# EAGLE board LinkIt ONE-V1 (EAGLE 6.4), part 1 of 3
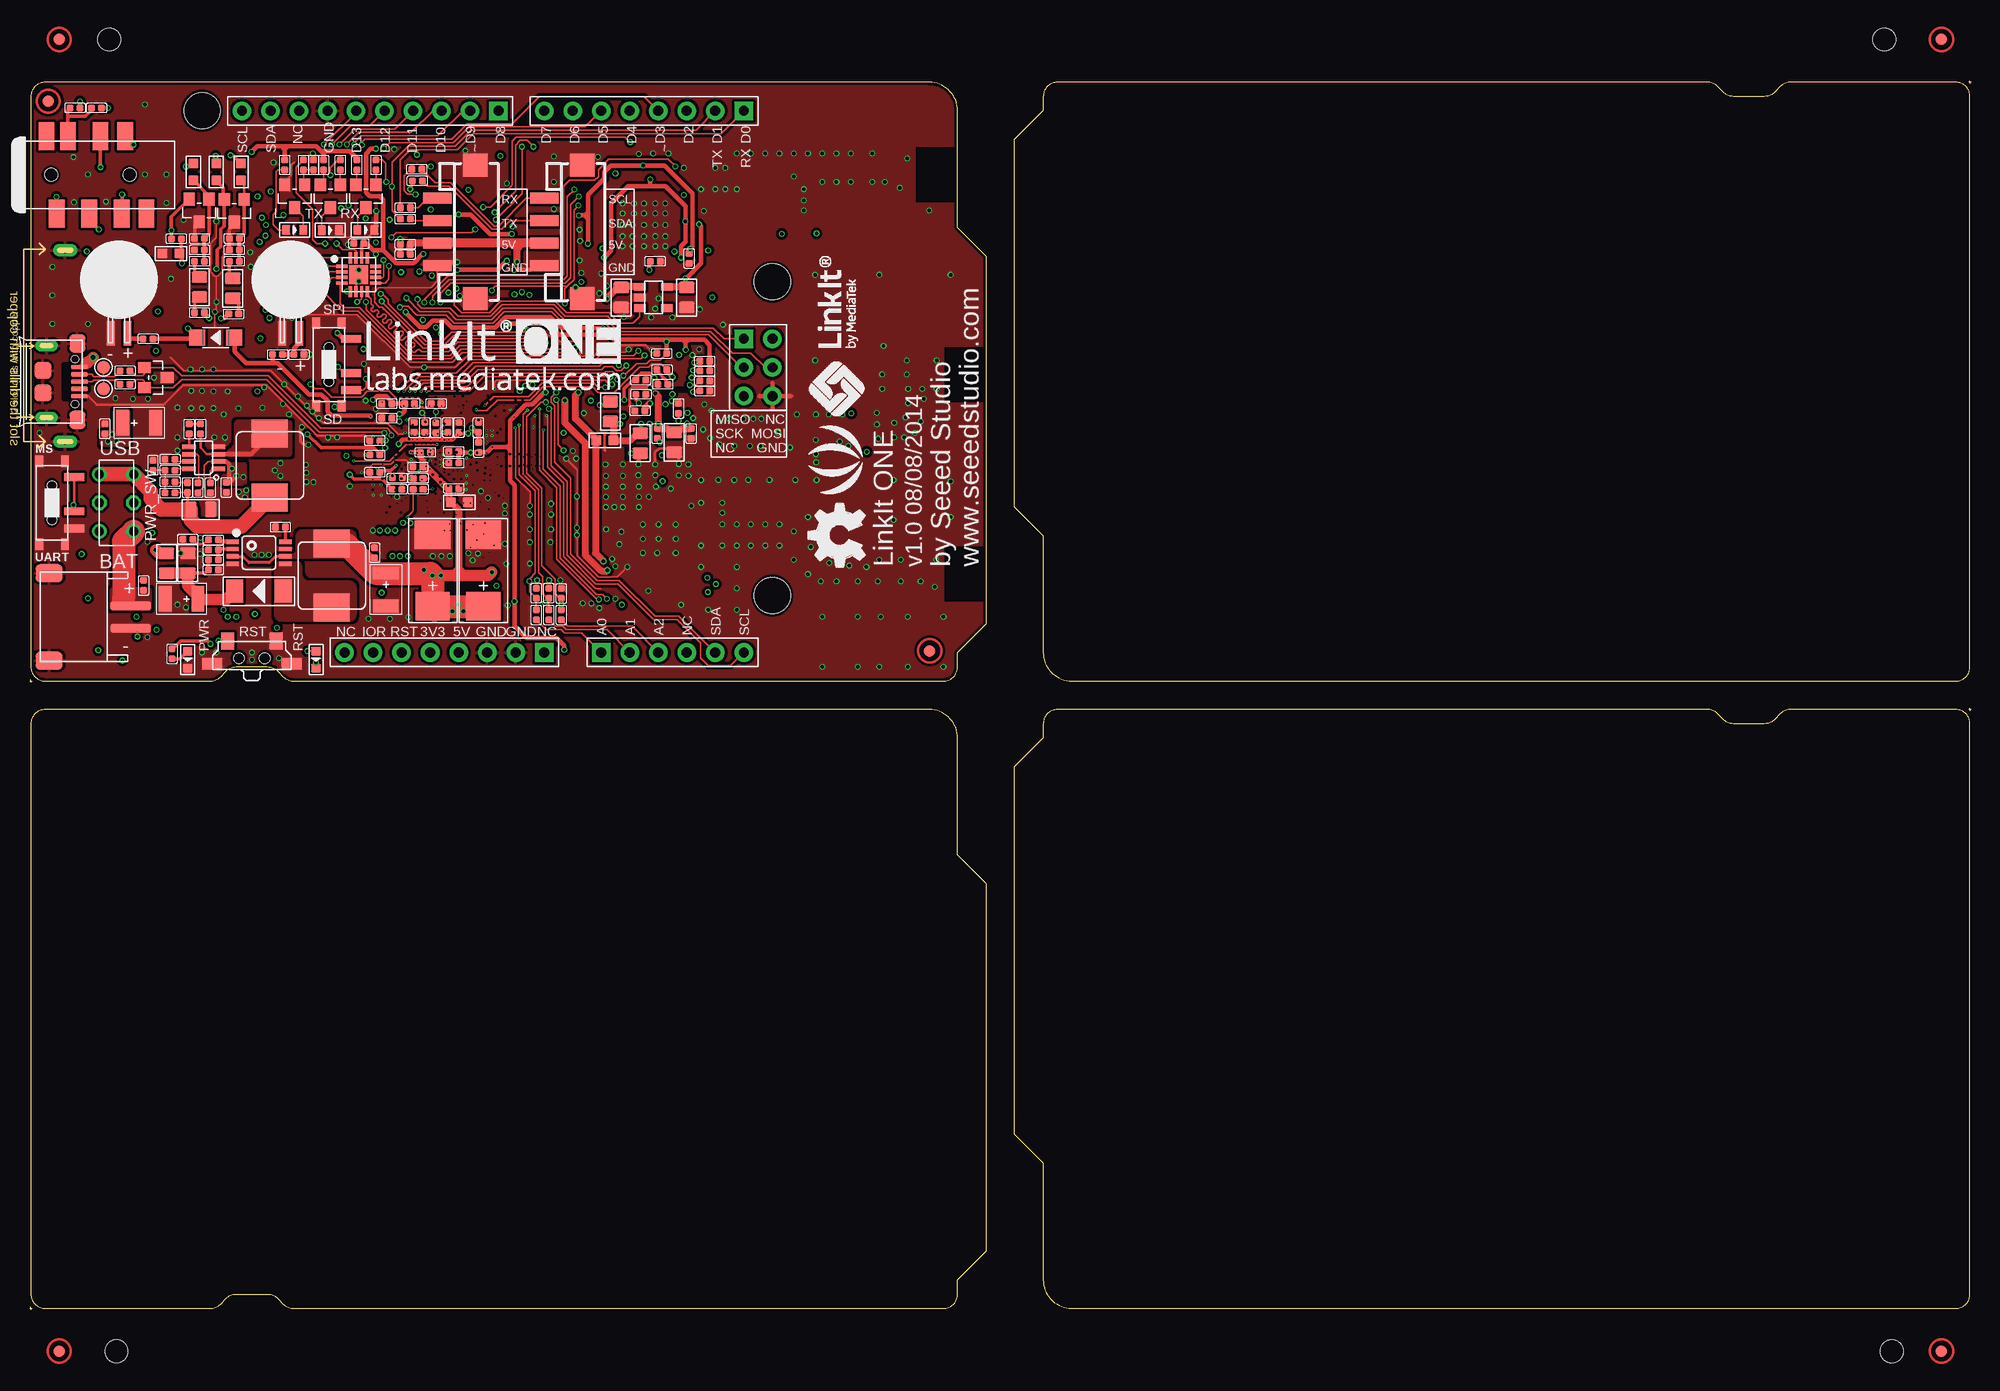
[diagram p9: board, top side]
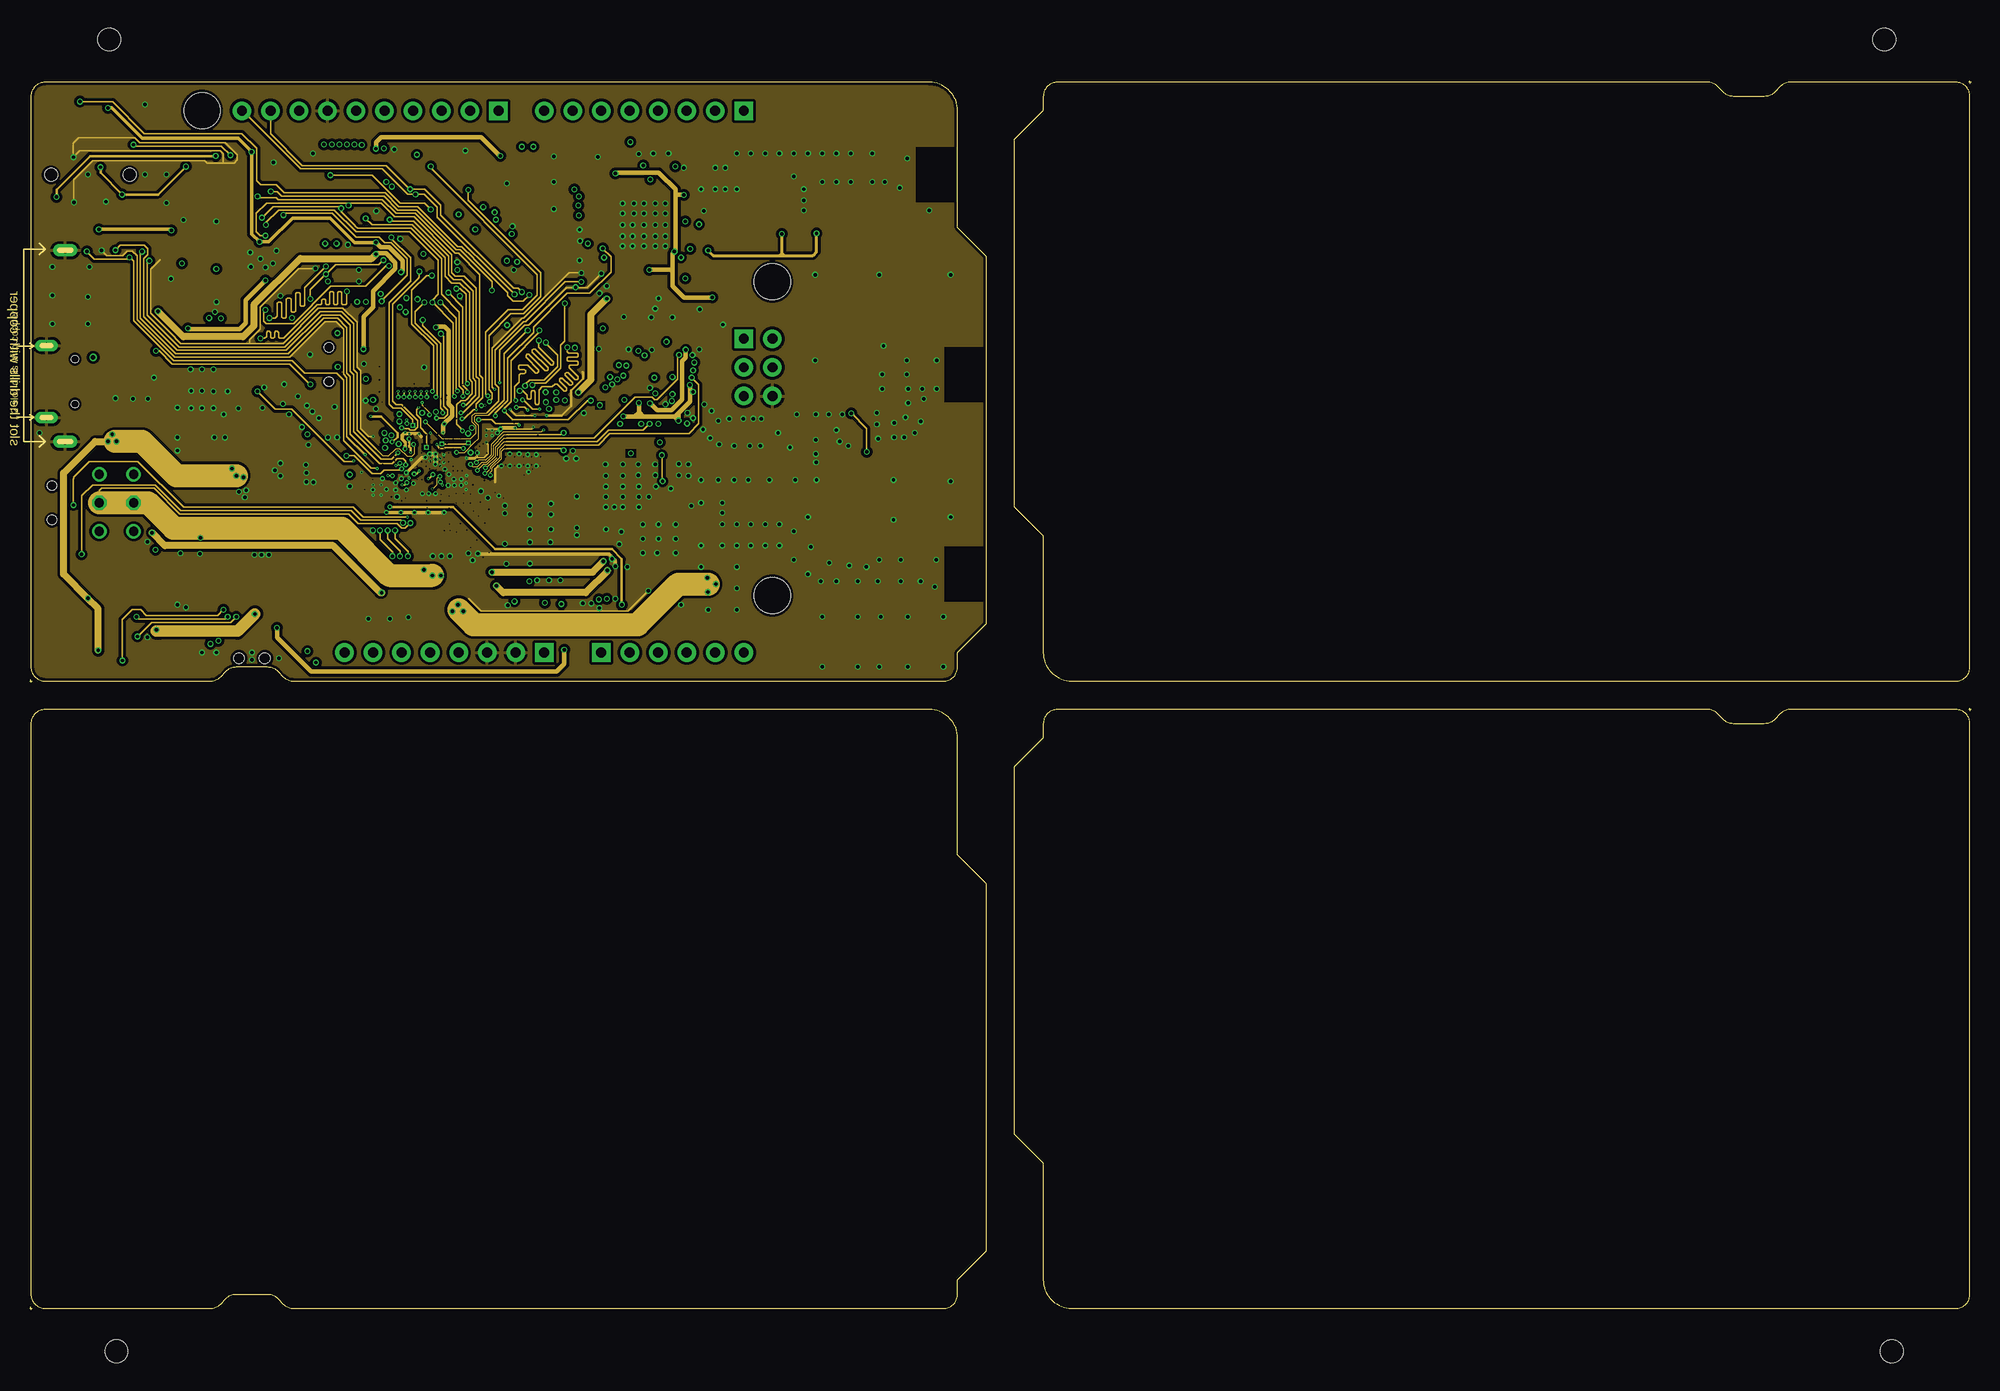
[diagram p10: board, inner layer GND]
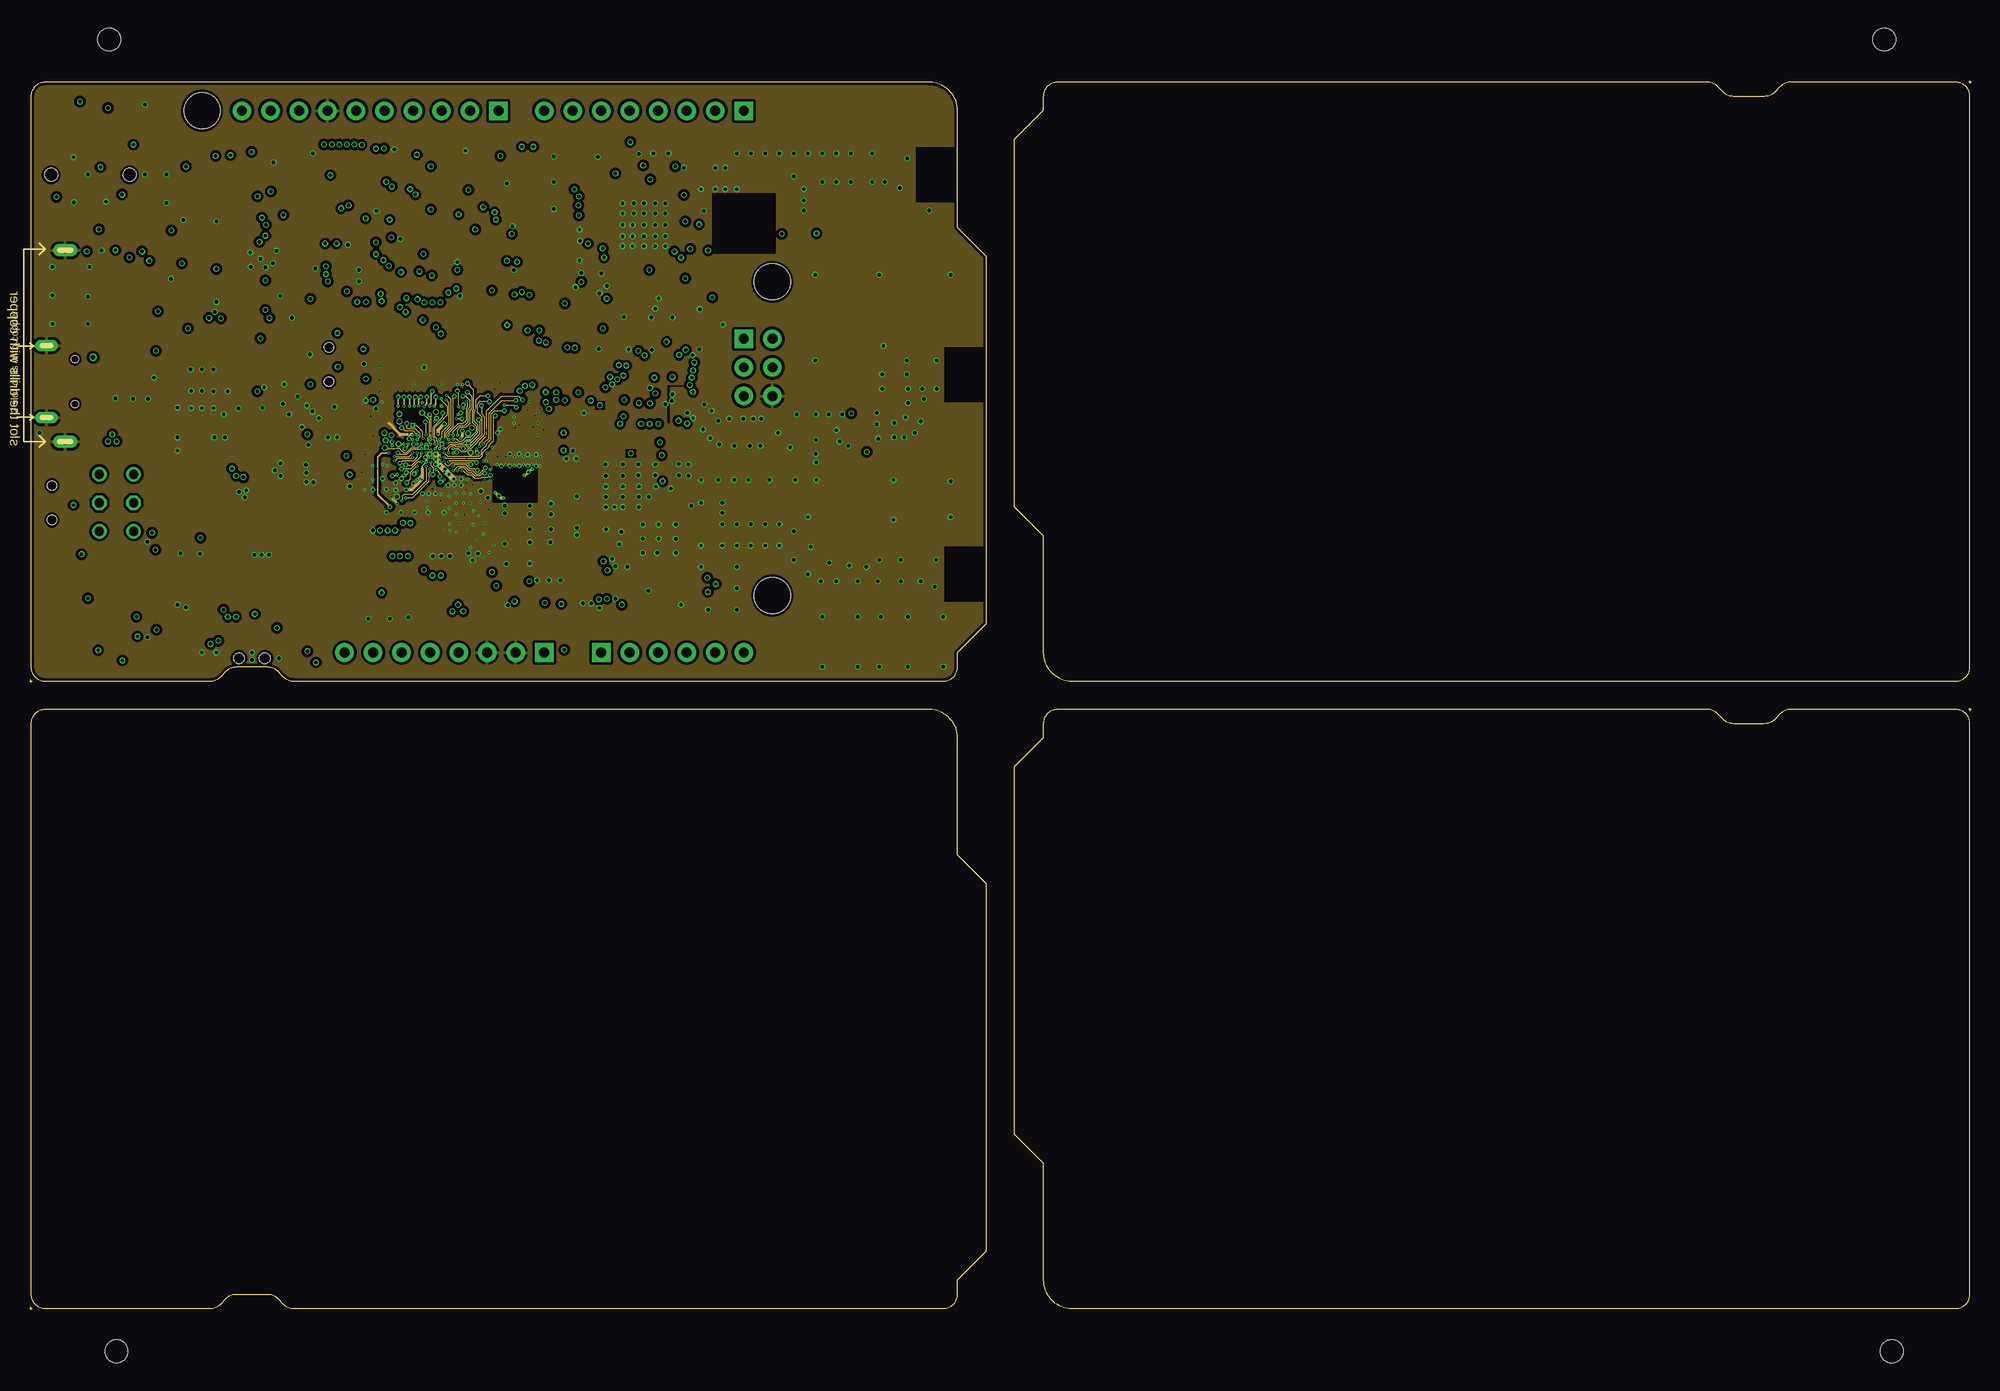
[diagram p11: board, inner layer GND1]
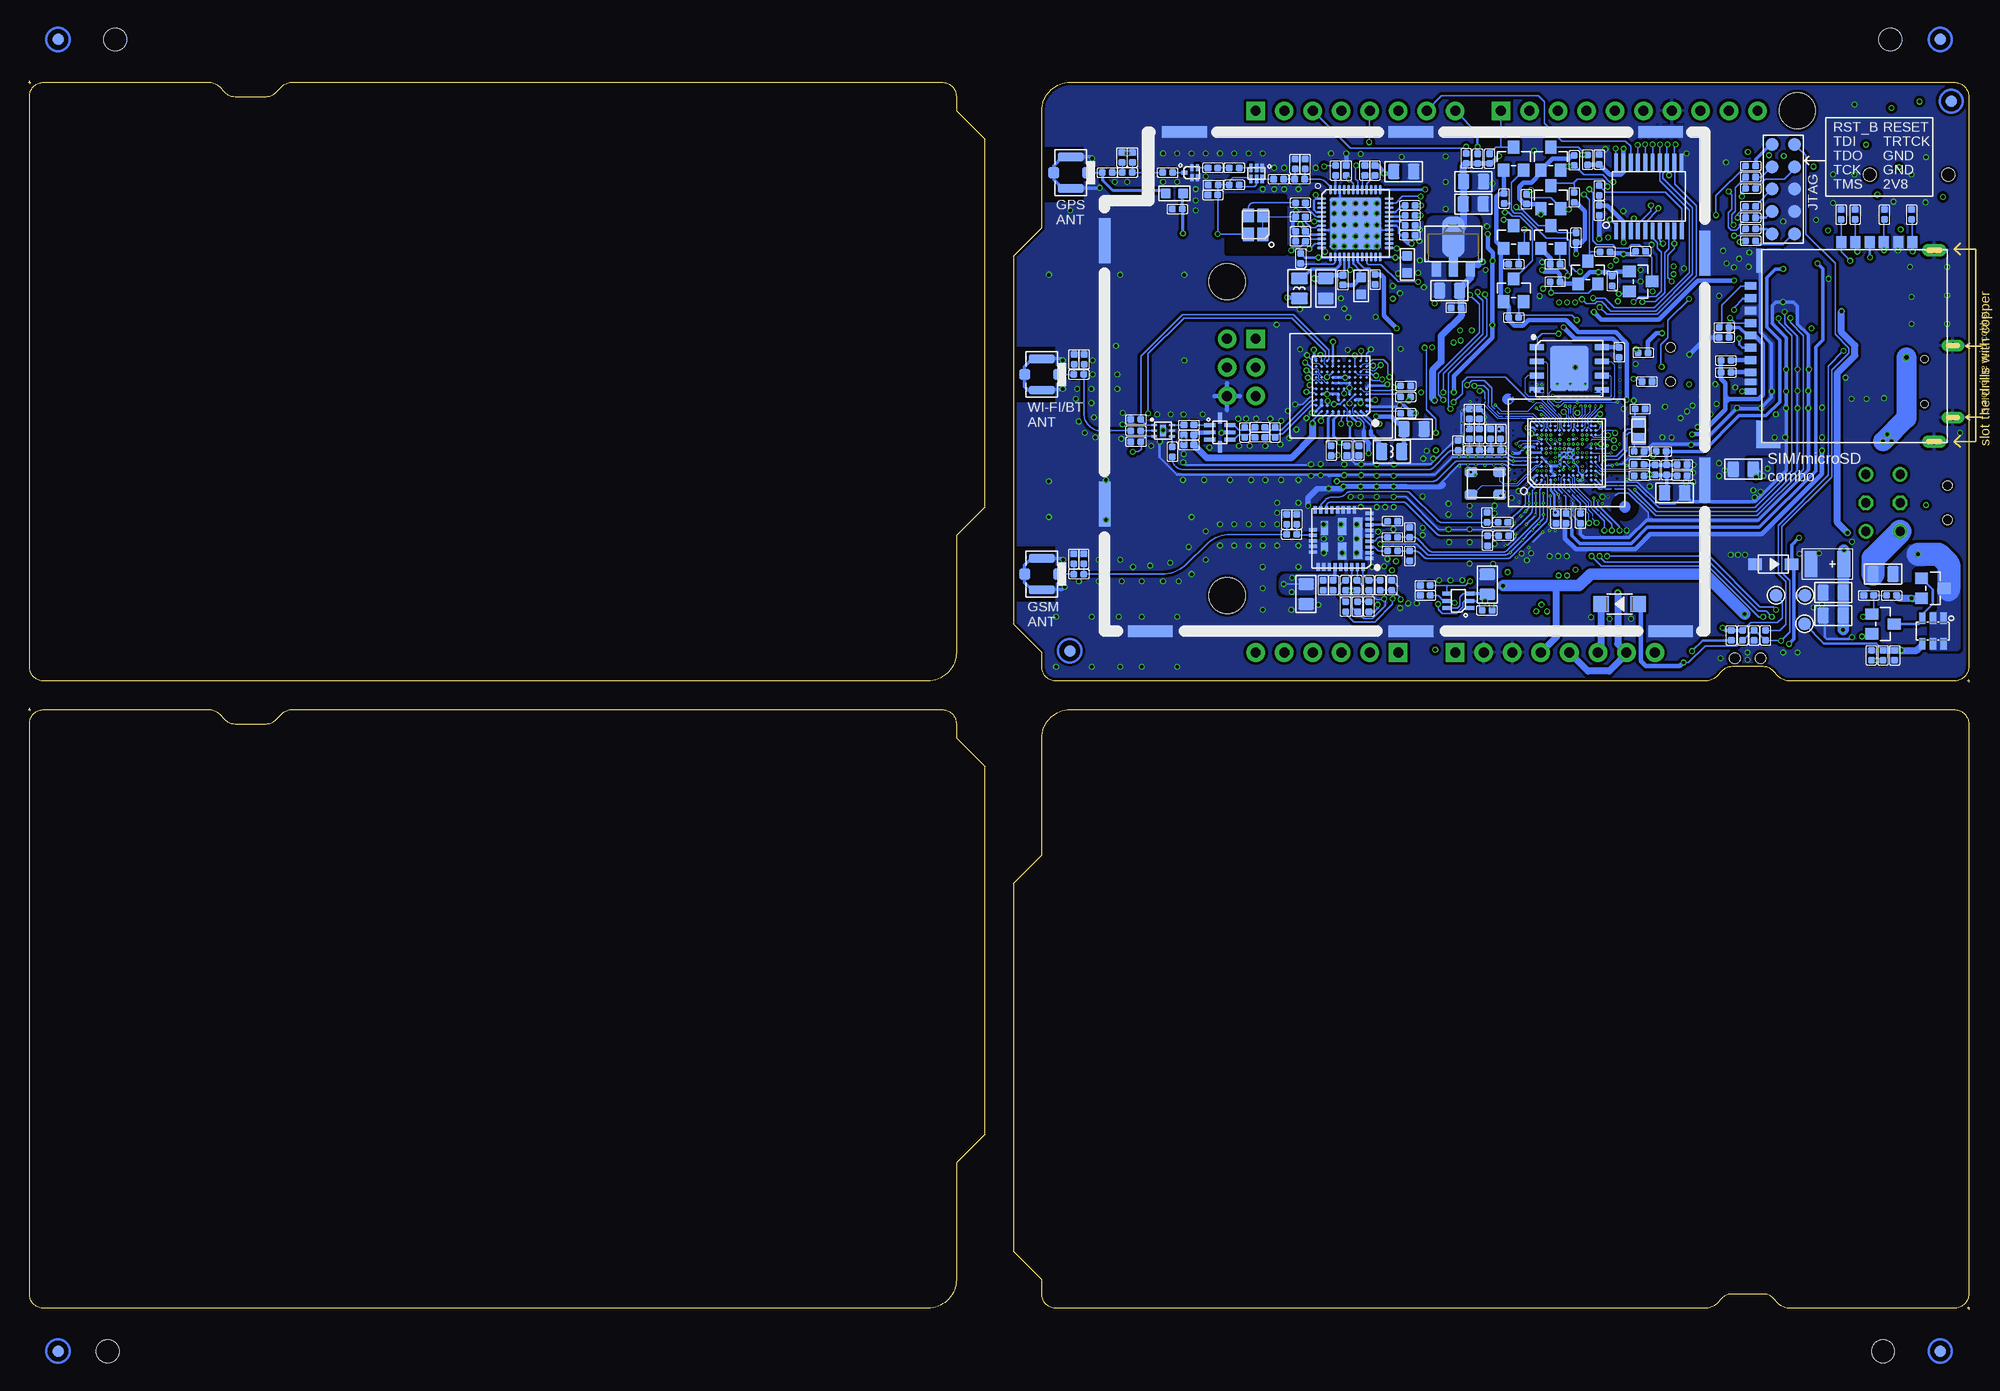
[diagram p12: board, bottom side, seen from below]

Size 172.97 x 109.47 mm. Coordinates in mm from the lower left corner, seen from the top.
Outline: 96 segments
Copper layers [2:(1+(2*15)+16):15]: Top 0.035mm / dielectric 0.2mm / GND 0.0175mm / dielectric 0.7mm / GND1 0.0175mm / dielectric 0.2mm / Bottom 0.035mm
Design rules "default *": minimum track width 3mil, minimum drill 4mil, track to track 3mil, track to pad 3mil, pad to pad 3mil, via to via 3mil, smd to smd 0mil, copper to edge 10mil, drill to drill 8mil, minimum pad ring 2mil, minimum via ring 2mil, stop-mask expansion 2mil, vias tented up to drill 25mil, thermal gap 10mil
Net classes: 0 default: width 0.076 mm, drill 0.102 mm, clearance 0.076 mm
Holes 2.03 mm at 7.11,113.16 165.23,113.16 165.86,-3.68 7.75,-3.68
tRestrict: area 53.2,75.8 to 55.1,76.8; area 56.4,80.4 to 56.9,80.9; area 57,81.3 to 57.5,81.8; area 58.4,79.6 to 58.9,80.1; area 50.5,80.4 to 52.5,81.4; area 65.4,80.6 to 67,82.2; 4 lines
bRestrict: area 61.1,94.1 to 66.2,99.2; area 41.4,72.1 to 45,75.1; area 53,75.8 to 54,76.8; area 57,81.3 to 57.5,81.8; area 55.8,80.3 to 58,81.8; area 65.4,80.6 to 67,82.2; 4 lines

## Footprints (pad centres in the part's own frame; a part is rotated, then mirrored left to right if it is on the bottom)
C0805 = smd 1.016 x 1.397: 1 -0.889,0; 2 0.889,0
C0402 = smd 0.635 x 0.635: 1 -0.445,0; 2 0.445,0
AVX-D = smd 2.54 x 3.048: + -3.175,0 | smd 2.54 x 3.175: - 3.175,0
C0603 = smd 0.889 x 0.889: 1 -0.762,0; 2 0.762,0
AVX-B = smd 1.143 x 2.286: + -1.46,0; - 1.46,0
2P-D6.8MMX1.8MMH = smd 2.2 x 0.7: + 4.8,0.75; - 4.8,-0.75
SOD123 = smd 1.397 x 1.397: + -1.651,0; - 1.651,0
SOD123-2.7X1.6 = smd 1.2 x 1.02: 1 -1.635,0; 2 1.635,0
SOT23 = smd 1.016 x 1.143: 1 -0.889,-1.016; 2 0.889,-1.016; 3 0,1.016
D2010 = smd 1.524 x 2.032: + -2.159,0; - 2.159,0
TP_4545 = smd 1.143 x 1.143: T 0,0
4P-U-FL = smd 1.016 x 1.016: D -1.524,0; GND3 1.524,0 | smd 2.286 x 0.762: GND1 0,1.397; GND2 0,-1.397
4P-SMD-2.0 = smd 0.965 x 2.54: 1 -3,0; 2 -1,0; 3 1,0; 4 3,0 | smd 2.032 x 2.184: SS1 -5.946,3.4; SS2 5.946,3.4
JST-SMD-2.0-90D = smd 1.6 x 2.4: 3 3.9,-2.181; 4 -3.9,-2.181 | smd 0.8 x 3.6: + -1,5.08; - 1,5.08
16P-L17.4MM*W16.5MM*H2.7MM = smd 0.7 x 1: 1 -2.35,9.25; 2 -1.25,9.25; 3 -0.15,9.25; 4 0.95,9.25; 5 2.05,9.25; 6 3.15,9.25; 7 4.25,9.25; 8 5.35,9.25 | smd 1.1 x 0.9: C1 9.25,-5.16; C2 9.25,-2.62; C3 9.25,-0.08; C5 9.25,-3.89; C6 9.25,-1.35; C7 9.25,1.19 | drill 0.5 pad 1.1 long: P1 -8.525,-7.1; P2 8.525,-7.1 | smd 0.5 x 1.65: P3 -8.85,7.425 | smd 2.45 x 0.5: P4 -7.875,8.5 | smd 2.13 x 0.5: P5 7.585,8.5 | smd 0.6 x 1: SA -4.05,9.25; SB -3.2,9.25
MICRO-USB = smd 0.381 x 1.524: 1 -1.3,-0.25; 2 -0.65,-0.25; 3 0,-0.25; 4 0.65,-0.25; 5 1.3,-0.25 | smd 1.6 x 1.397: S1 -3.4,-0.427; S6 3.4,-0.427 | drill 0.508 pad 1.016 long: S2 -3.226,-3.175; S5 3.226,-3.175 | smd 1.5 x 1.5: S3 -1,-3.5; S4 1,-3.5 | hole 0.635: -2,-0.65; 2,-0.65
8P-3.5-SMD = smd 1.4 x 2.5: 1 2.8,-3.45; 2 5.7,-3.45; 3 8.6,-3.45; 4 8.9,3.45; 5 1.9,3.45; 6 3.8,3.45; 7 6.7,3.45; 8 10.8,-3.45 | hole 1.149: 2.3,0; 9.3,0
2*5P-2.0-TESTPOINT = smd 1.143 x 1.143: 1 -1,4; 2 -1,2; 3 -1,0; 4 -1,-2; 5 -1,-4; 6 1,-4; 7 1,-2; 8 1,0; 9 1,2; 10 1,4
LED-0603 = smd 0.762 x 0.889: + -0.762,0; - 0.762,0
L0402 = smd 0.635 x 0.635: 1 -0.445,0; 2 0.445,0
L0603 = smd 0.889 x 0.889: 1 -0.762,0; 2 0.762,0
0806 = smd 1.016 x 1.524: 1 -0.889,0; 2 0.889,0
L0630 = smd 2.5 x 3.2: 1 -2.85,0; 2 2.85,0
L0805 = smd 1.016 x 1.397: 1 -0.889,0; 2 0.889,0
ROUND-MARK-1.0 = smd 1.016 x 1.016: P$1 0,0
R0402 = smd 0.635 x 0.635: 1 -0.445,0; 2 0.445,0
R0805 = smd 1.016 x 1.397: 1 -0.889,0; 2 0.889,0
4P-SMD-7X3.5X3.5H = smd 1.143 x 1.524: 1 -2.159,1.524; 2 2.159,1.524 | smd 1.778 x 1.016: S1 -3.556,-0.508; S2 3.556,-0.508 | hole 0.95: -1.15,0; 1.15,0
3P-SMD-2CH-6.6X2.8-REINFORCE = smd 1.8 x 0.7: A 1.978,2.286; B 1.978,-2.286; COM 1.978,-0.762 | smd 0.7 x 1.016: SS1 -1.15,-3.683; SS2 1.15,-3.683; SS3 1.15,3.683; SS4 -1.15,3.683 | hole 0.813: 0,-1.524; 0,1.524
6P-2CH-2.54-7.6X3.0 = drill 0.813 pad 1.27: CH1A -1.524,2.54; CH1B -1.524,-2.54; CH2A 1.524,2.54; CH2B 1.524,-2.54 | drill 0.813 pad 1.27 octagon: COM1 -1.524,0; COM2 1.524,0
TFBGA84 = smd 0.25 x 0.25: A1 -2.25,2.25; A2 -1.75,2.25; A3 -1.25,2.25; A4 -0.75,2.25; A5 -0.25,2.25; A6 0.25,2.25; A7 0.75,2.25; A8 1.25,2.25; A9 1.75,2.25; A10 2.25,2.25; B1 -2.25,1.75; B3 -1.25,1.75; B5 -0.25,1.75; B8 1.25,1.75; B9 1.75,1.75; B10 2.25,1.75; C1 -2.25,1.25; C2 -1.75,1.25; C3 -1.25,1.25; C5 -0.25,1.25; C6 0.25,1.25; C9 1.75,1.25; C10 2.25,1.25; D1 -2.25,0.75; D2 -1.75,0.75; D3 -1.25,0.75; D4 -0.75,0.75; D6 0.25,0.75; D7 0.75,0.75; D9 1.75,0.75; D10 2.25,0.75; E1 -2.25,0.25; E2 -1.75,0.25; E3 -1.25,0.25; E5 -0.25,0.25; E6 0.25,0.25; E7 0.75,0.25; E8 1.25,0.25; E9 1.75,0.25; E10 2.25,0.25; F2 -1.75,-0.25; F3 -1.25,-0.25; F4 -0.75,-0.25; F6 0.25,-0.25; F7 0.75,-0.25; F8 1.25,-0.25; F9 1.75,-0.25; F10 2.25,-0.25; G1 -2.25,-0.75; G2 -1.75,-0.75; G3 -1.25,-0.75; G4 -0.75,-0.75; G6 0.25,-0.75; G7 0.75,-0.75; G9 1.75,-0.75; G10 2.25,-0.75; H1 -2.25,-1.25; H2 -1.75,-1.25; H3 -1.25,-1.25; H4 -0.75,-1.25; H5 -0.25,-1.25; H6 0.25,-1.25; H7 0.75,-1.25; H8 1.25,-1.25; H9 1.75,-1.25; H10 2.25,-1.25; J1 -2.25,-1.75; J2 -1.75,-1.75; J3 -1.25,-1.75; J4 -0.75,-1.75; J5 -0.25,-1.75; J6 0.25,-1.75; J7 0.75,-1.75; J8 1.25,-1.75; J9 1.75,-1.75; J10 2.25,-1.75; K1 -2.25,-2.25; K2 -1.75,-2.25; K4 -0.75,-2.25; K6 0.25,-2.25; K7 0.75,-2.25; K8 1.25,-2.25; K9 1.75,-2.25; K10 2.25,-2.25
QFN48-6X6MM = smd 0.25 x 0.8: 1 -2.2,-3; 2 -1.8,-3; 3 -1.4,-3; 4 -1,-3; 5 -0.6,-3; 6 -0.2,-3; 7 0.2,-3; 8 0.6,-3; 9 1,-3; 10 1.4,-3; 11 1.8,-3; 12 2.2,-3; 25 2.2,3; 26 1.8,3; 27 1.4,3; 28 1,3; 29 0.6,3; 30 0.2,3; 31 -0.2,3; 32 -0.6,3; 33 -1,3; 34 -1.4,3; 35 -1.8,3; 36 -2.2,3 | smd 0.8 x 0.25: 13 3,-2.2; 14 3,-1.8; 15 3,-1.4; 16 3,-1; 17 3,-0.6; 18 3,-0.2; 19 3,0.2; 20 3,0.6; 21 3,1; 22 3,1.4; 23 3,1.8; 24 3,2.2; 37 -3,2.2; 38 -3,1.8; 39 -3,1.4; 40 -3,1; 41 -3,0.6; 42 -3,0.2; 43 -3,-0.2; 44 -3,-0.6; 45 -3,-1; 46 -3,-1.4; 47 -3,-1.8; 48 -3,-2.2 | smd 4.6 x 4.6: PAD 0,0
WSON8-6X5X0.8H-W/HEAT = smd 0.5 x 1.25: 1 -1.905,-2.875; 2 -0.635,-2.875; 3 0.635,-2.875; 4 1.905,-2.875; 5 1.905,2.875; 6 0.635,2.875; 7 -0.635,2.875; 8 -1.905,2.875 | smd 4 x 3.4: PAD 0,0
SOT-25J = smd 0.7 x 1: 1 -0.95,-1.2; 2 0,-1.2; 3 0.95,-1.2; 4 0.95,1.2; 5 -0.95,1.2
TQFN16 = smd 1 x 0.3: 1 -1.5,0.75; 2 -1.5,0.25; 3 -1.5,-0.25; 4 -1.5,-0.75; 9 1.5,-0.75; 10 1.5,-0.25; 11 1.5,0.25; 12 1.5,0.75 | smd 0.3 x 1: 5 -0.75,-1.5; 6 -0.25,-1.5; 7 0.25,-1.5; 8 0.75,-1.5; 13 0.75,1.5; 14 0.25,1.5; 15 -0.25,1.5; 16 -0.75,1.5 | smd 1.7 x 1.7: PAD 0,0
VFBGA143 = smd 0.25 x 0.25: A1 -2.4,2.6; A2 -2,2.6; A3 -1.6,2.6; A5 -0.8,2.6; A6 -0.4,2.6; A8 0.4,2.6; A9 0.8,2.6; A11 1.6,2.6; A12 2,2.6; A13 2.4,2.6; B1 -2.4,2.2; B2 -2,2.2; B3 -1.6,2.2; B4 -1.2,2.2; B5 -0.8,2.2; B6 -0.4,2.2; B7 0,2.2; B8 0.4,2.2; B9 0.8,2.2; B10 1.2,2.2; B11 1.6,2.2; B12 2,2.2; B13 2.4,2.2; C2 -2,1.8; C3 -1.6,1.8; C4 -1.2,1.8; C5 -0.8,1.8; C7 0,1.8; C8 0.4,1.8; C11 1.6,1.8; C12 2,1.8; D1 -2.4,1.4; D2 -2,1.4; D3 -1.6,1.4; D4 -1.2,1.4; D5 -0.8,1.4; D7 0,1.4; D8 0.4,1.4; D10 1.2,1.4; D11 1.6,1.4; D12 2,1.4; D13 2.4,1.4; E1 -2.4,1; E2 -2,1; E5 -0.8,1; E6 -0.4,1; E7 0,1; E8 0.4,1; E9 0.8,1; E12 2,1; E13 2.4,1; F2 -2,0.6; F3 -1.6,0.6; F4 -1.2,0.6; F5 -0.8,0.6; F6 -0.4,0.6; F7 0,0.6; F8 0.4,0.6; F9 0.8,0.6; F10 1.2,0.6; F11 1.6,0.6; F12 2,0.6; G1 -2.4,0.2; G2 -2,0.2; G4 -1.2,0.2; G5 -0.8,0.2; G6 -0.4,0.2; G7 0,0.2; G8 0.4,0.2; G9 0.8,0.2; G12 2,0.2; G13 2.4,0.2; H1 -2.4,-0.2; H2 -2,-0.2; H5 -0.8,-0.2; H6 -0.4,-0.2; H7 0,-0.2; H8 0.4,-0.2; H9 0.8,-0.2; H10 1.2,-0.2; H12 2,-0.2; H13 2.4,-0.2; J2 -2,-0.6; J3 -1.6,-0.6; J4 -1.2,-0.6; J5 -0.8,-0.6; J6 -0.4,-0.6; J7 0,-0.6; J8 0.4,-0.6; J9 0.8,-0.6; J10 1.2,-0.6; J11 1.6,-0.6; J12 2,-0.6; K1 -2.4,-1; K2 -2,-1; K5 -0.8,-1; K6 -0.4,-1; K7 0,-1; K8 0.4,-1; K9 0.8,-1; K12 2,-1; K13 2.4,-1; L1 -2.4,-1.4; L2 -2,-1.4; L3 -1.6,-1.4; L4 -1.2,-1.4; L6 -0.4,-1.4; L7 0,-1.4; L9 0.8,-1.4; L10 1.2,-1.4; L11 1.6,-1.4; L12 2,-1.4; L13 2.4,-1.4; M2 -2,-1.8; M3 -1.6,-1.8; M6 -0.4,-1.8; M7 0,-1.8; M10 1.2,-1.8; M11 1.6,-1.8; M12 2,-1.8; N1 -2.4,-2.2; N2 -2,-2.2; N3 -1.6,-2.2; N4 -1.2,-2.2; N5 -0.8,-2.2; N6 -0.4,-2.2; N7 0,-2.2; N8 0.4,-2.2; N9 0.8,-2.2; N10 1.2,-2.2; N11 1.6,-2.2; N12 2,-2.2; N13 2.4,-2.2; P1 -2.4,-2.6; P2 -2,-2.6; P3 -1.6,-2.6; P5 -0.8,-2.6; P6 -0.4,-2.6; P8 0.4,-2.6; P9 0.8,-2.6; P11 1.6,-2.6; P12 2,-2.6; P13 2.4,-2.6
SOT23-6L = smd 0.55 x 1.016: 1 -0.95,-1.143; 2 0,-1.143; 3 0.95,-1.143; 4 0.95,1.143; 5 0,1.143; 6 -0.95,1.143
5P-SMD-1.4X1.1MM = smd 0.55 x 0.326: 1 -0.65,0 | smd 0.25 x 0.625: 2 0,-0.438; 3 0.5,-0.438; 4 0.5,0.438; 5 0,0.438
SHIELD-SMD-44.5X53.5 = smd 4 x 1.016: 1 3.937,0; 4 49.403,44.45; 5 46.355,0; 6 3.048,44.45; 9 26.162,44.45; 10 26.162,0 | smd 1.016 x 4: 2 0,30.988; 3 53.467,9.652; 7 53.467,33.147; 8 0,10.795
ARDUINO-38P = drill 0.889 pad 1.651 square: 1 63.5,50.8; 9 41.656,50.8; 19 50.8,2.54; 25 45.72,2.54; 38 63.5,30.48 | drill 0.889 pad 1.651: 2 60.96,50.8; 3 58.42,50.8; 4 55.88,50.8; 5 53.34,50.8; 6 50.8,50.8; 7 48.26,50.8; 8 45.72,50.8; 10 39.116,50.8; 11 36.576,50.8; 12 34.036,50.8; 13 31.496,50.8; 14 28.956,50.8; 15 26.416,50.8; 16 23.876,50.8; 17 21.336,50.8; 18 18.796,50.8; 20 53.34,2.54; 21 55.88,2.54; 22 58.42,2.54; 23 60.96,2.54; 24 63.5,2.54; 26 43.18,2.54; 27 40.64,2.54; 28 38.1,2.54; 29 35.56,2.54; 30 33.02,2.54; 31 30.48,2.54; 32 27.94,2.54; 33 66.04,30.48; 34 66.04,27.94; 35 66.04,25.4; 36 63.5,25.4; 37 63.5,27.94 | hole 3.2: 15.24,50.8; 66.04,35.56; 66.04,7.62
TSOT23-8 = smd 0.4 x 1.2: 1 -0.975,-1.3; 2 -0.325,-1.3; 3 0.325,-1.3; 4 0.975,-1.3; 5 0.975,1.3; 6 0.325,1.3; 7 -0.325,1.3; 8 -0.975,1.3
6P-SMD-1.5X1.0X0.72H = smd 0.3 x 0.75: 1 -0.5,-0.5; 2 0,-0.5; 3 0.5,-0.5; 4 0.5,0.5; 5 0,0.5; 6 -0.5,0.5
32P-SMD-RF1798-5.3MMX5.25MMX0.73H = smd 0.7 x 0.3: 1 -2.525,1.77; 2 -2.525,1.27; 3 -2.525,0.77; 4 -2.525,0.27; 5 -2.525,-0.23; 6 -2.525,-0.73; 7 -2.525,-1.23; 8 -2.525,-1.73; 9 -2.525,-2.23; 18 2.525,-0.785; 19 2.525,-0.285; 20 2.525,0.215; 21 2.525,0.715; 22 2.525,1.215 | smd 0.3 x 0.7: 10 -1.175,-2.55; 11 -0.675,-2.55; 12 -0.175,-2.55; 13 0.325,-2.55; 14 0.825,-2.55; 15 1.325,-2.55; 16 1.825,-2.55; 17 2.325,-2.55; 23 2.055,2.55; 24 1.555,2.55; 25 1.055,2.55; 26 0.555,2.55; 27 0.055,2.55; 28 -0.445,2.55; 29 -0.945,2.55; 30 -1.445,2.55; 31 -1.945,2.55 | smd 0.805 x 3.715: 32 -1.473,0 | smd 0.785 x 1.535: 33 -0.083,1.133; 34 -0.083,-1.055 | smd 0.635 x 0.8: 35 1.493,0.765 | smd 0.635 x 1.245: 36 1.493,-0.933
8P-SMD-2X1.25X0.7H = smd 0.35 x 1: 1 0.65,0.9; 2 0,0.9; 3 -0.65,0.9; 5 -0.65,-0.9; 6 0,-0.9; 7 0.65,-0.9 | smd 1 x 0.35: 4 -1.281,0; 8 1.281,0
TSON6 = smd 0.5 x 0.2: 1 -0.8,0.5; 2 -0.8,0; 3 -0.8,-0.5; 4 0.8,-0.5; 5 0.8,0; 6 0.8,0.5 | smd 0.5 x 1: PAD 0,0
SOT363 = smd 0.35 x 0.8: 1 -0.65,-1.025; 2 0,-1.025; 3 0.65,-1.025; 4 0.65,1.025; 5 0,1.025; 6 -0.65,1.025
TSSOP20 = smd 0.35 x 1.5: 1 -2.925,-3.065; 2 -2.275,-3.065; 3 -1.625,-3.065; 4 -0.975,-3.065; 5 -0.325,-3.065; 6 0.325,-3.065; 7 0.975,-3.065; 8 1.625,-3.065; 9 2.275,-3.065; 10 2.925,-3.065; 11 2.91,3.065; 12 2.26,3.065; 13 1.61,3.065; 14 0.96,3.065; 15 0.325,3.065; 16 -0.325,3.065; 17 -0.975,3.065; 18 -1.625,3.065; 19 -2.275,3.065; 20 -2.925,3.065
SOT89 = smd 0.8 x 1.4: 1 -1.524,-1.905; 3 1.524,-1.905 | smd 0.8 x 1.9: 2 0,-1.651 | smd 2.032 x 3.65: 4 0,0.94
MSOP8 = smd 0.4 x 1.1: 1 -0.975,-2.35; 2 -0.325,-2.35; 3 0.325,-2.35; 4 0.975,-2.35; 5 0.975,2.35; 6 0.325,2.35; 7 -0.325,2.35; 8 -0.975,2.35
2P-SMD-2.05X1.2 = smd 1 x 1.25: 1 -0.75,0; 2 0.75,0
2520 = smd 1.2 x 1: 1 -0.85,-0.65; 2 0.85,-0.65; 3 0.85,0.65; 4 -0.85,0.65
4P-SMD-3.2X2.5 = smd 1.143 x 0.889: 1 -1.27,-1.016; 2 1.27,-1.016; 3 1.27,1.016; 4 -1.27,1.016

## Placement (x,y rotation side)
C1  4.7uF  [C0805]  46.36,90.78 180 bottom
C2  4.7uF  [C0805]  44.22,100.51 0 bottom
C3  100nF  [C0402]  30.73,67.44 90 top
C4  100nF  [C0402]  16.38,65.91 0 top
C5  100nF  [C0402]  33.02,97.92 270 bottom
C6  1uF  [C0402]  50.27,79.86 0 bottom
C7  100nF  [C0402]  33.02,102.46 90 bottom
C8  1uF  [C0402]  37.8,73.15 0 top
C9  1uF  [C0402]  36.2,78.56 270 top
C10  1uF  [C0402]  31.83,79.43 180 top
C11  4.7uF  [C0805]  49.53,78.46 0 bottom
C12  4.7uF  [C0805]  54.41,77.19 270 top
C13  1uF  [C0402]  54.47,81.55 180 top
C14  100nF  [C0402]  54.38,80.09 0 top
C15  1uF  [C0402]  55.5,76.53 270 bottom
C16  1uF  [C0402]  60.15,82.73 180 top
C17  18pF  [C0402]  60.15,81.84 180 top
C18  100nF  [C0402]  58.93,78.05 90 top
C19  100nF  [C0402]  57.81,80.29 270 top
C20  1nF  [C0402]  56.9,76.53 90 bottom
C21  100nF  [C0402]  56.41,82.45 0 top
C22  1uF  [C0402]  54.44,82.83 0 top
C23  1uF  [C0402]  56.31,85.19 180 top
C24  18pF  [C0402]  71.48,101.3 180 bottom
C25  18pF  [C0402]  67.44,101.73 0 bottom
C26  1uF  [C0402]  59.64,95.17 180 bottom
C27  DNP/18pF  [C0402]  75.54,102.64 90 bottom
C28  100nF  [C0402]  33.48,94.92 180 top
C29  1uF  [C0402]  52.98,91.77 270 bottom
C30  SMD CAP Tantalum 470uF-6.3V;D  [AVX-D]  35.92,65.84 90 top
C31  220nF  [C0402]  55.85,91.72 90 bottom
C32  22uF  [C0805]  44.25,98.5 0 bottom
C33  SMD CAP Tantalum 470uF-6.3V;D  [AVX-D]  40.44,65.84 90 top
C34  4.7uF  [C0805]  50.44,101.4 0 bottom
C35  4.7uF  [C0805]  57.38,90.98 270 bottom
C36  1uF  [C0402]  58.75,93.65 270 top
C37  1uF  [C0402]  59.61,93.65 270 bottom
C38  1uF  [C0402]  59.64,97.36 180 bottom
C39  1uF  [C0402]  59.64,96.06 180 bottom
C40  100nF  [C0402]  49.89,95.71 0 bottom
C41  2.2uF  [C0603]  50.11,93.12 270 bottom
C42  DNP/100nF  [C0402]  55.55,101.47 90 bottom
C43  1nF  [C0402]  59.64,98.6 180 bottom
C44  100nF  [C0402]  55.73,93.4 0 top
C45  4.7uF  [C0805]  52.71,90.17 270 top
C46  4.7uF  [C0805]  58.55,90.17 270 top
C47  1uF  [C0402]  37.26,78.59 90 top
C48  1uF  [C0402]  9.02,63.63 180 bottom
C49  SMD CAP Tantalum 47uF-10V;B  [AVX-B]  9.78,78.99 0 top
C50  SMD CAP Tantalum 47uF-10V;B  [AVX-B]  31.75,64.16 270 top
C51  22uF  [C0805]  18.11,90.98 90 top
C52  22uF  [C0805]  15.14,91.11 90 top
C53  390pF  [C0402]  15.14,94.41 180 top
C54  390pF  [C0402]  18.24,94.41 180 top
C55  100nF  [C0402]  29.46,74.3 0 bottom
C56  33pF  [C0402]  25.63,75.29 0 bottom
C57  33pF  [C0402]  25.63,74.3 0 bottom
C58  100nF  [C0402]  29.46,75.31 0 bottom
C59  100pF  [C0402]  28.07,74.8 270 bottom
C60  4.7uF  [C0805]  26.31,72.77 0 bottom
C61  27pF  [C0402]  7.62,97.56 90 bottom
C62  27pF  [C0402]  10.24,97.56 90 bottom
C63  1uF  [C0402]  37.8,76.45 180 top
C64  27pF  [C0402]  11.48,97.56 90 bottom
C65  1uF  [C0402]  5.21,97.56 90 bottom
C66  100nF  [C0402]  21.89,86.61 180 bottom
C67  1.2pF  [C0402]  59.69,100.71 0 bottom
C68  DNP/18pF  [C0402]  60.12,102.06 90 bottom
C69  1uF  [C0402]  38.25,78.59 90 top
C70  1uF  [C0402]  31.83,80.72 180 top
C71  1uF  [C0402]  37.8,75.44 180 top
C72  1uF  [C0402]  35.26,76.38 0 top
C73  2.2uF  [C0603]  38.3,71.93 0 top
C74  22uF  [C0805]  20.19,74.87 180 bottom
C75  22pF  [C0402]  29.39,80.24 0 bottom
C76  22pF  [C0402]  29.46,76.45 0 bottom
C77  100nF  [C0402]  12.52,75.77 180 top
C78  15pF  [C0402]  14.08,73.24 270 top
C79  22uF  [C0805]  15.27,71.3 0 top
C80  18pF  [C0402]  70.61,98.04 180 bottom
C81  330pF  [C0402]  19.23,60.07 270 bottom
C82  DNP/18pF  [C0402]  59.97,70.41 90 bottom
C83  DNP/18pF  [C0402]  60.86,70.41 90 bottom
C84  1.2pF  [C0402]  79.81,84.66 90 bottom
C85  18pF  [C0402]  76.83,101.3 180 bottom
C87  100nF  [C0402]  29.34,94.97 180 top
C88  SMD CAP Tantalum 47uF-10V;B  [AVX-B]  13.54,63.32 180 top
C89  DNP/22pF  [C0402]  47.37,63.8 90 top
C90  100nF  [C0402]  33.48,94.01 180 top
C91  1uF  [C0402]  31.24,85.29 270 bottom
C92  1uF  [C0402]  34.7,70.48 270 bottom
C93  1uF  [C0402]  24,85.09 0 top
C94  1uF  [C0402]  32.77,74.09 0 top
C95  1uF  [C0402]  30.76,76.15 180 top
C96  1uF  [C0402]  30.76,77.42 180 top
C97  100nF  [C0402]  30.76,74.6 180 top
C98  1uF  [C0402]  6.71,78.49 90 top
C99  2.2uF  [C0603]  54.23,91.21 270 bottom
C100  22nF  [C0402]  16.1,73.23 270 top
C101  100nF  [C0402]  34.59,75.08 180 top
C102  DNP/22pF  [C0402]  46.25,63.83 90 top
C103  DNP/22pF  [C0402]  48.51,64.52 180 bottom
C104  1uF  [C0402]  36.88,70.48 270 bottom
C105  100nF  [C0402]  15.24,78.46 90 top
C106  100nF  [C0402]  17.53,73.25 270 top
C107  DNP/EECENOF204Rk  [2P-D6.8MMX1.8MMH]  23.27,91.77 270 top
C108  100nF  [C0402]  45.77,89.26 180 bottom
C109  1uF  [C0402]  10.16,64.52 90 top
C110  1.2pF  [C0402]  45.61,77 90 bottom
C111  1.5pF  [C0402]  44.59,78.02 90 bottom
C112  1.8pF  [C0402]  43.7,79.79 90 bottom
C113  1.5pF  [C0402]  42.68,78.02 90 bottom
C114  0.5pF  [C0402]  41.8,78.02 90 bottom
C115  1.2pF  [C0402]  78.92,84.66 90 bottom
C116  1uF  [C0402]  6.71,58.29 270 bottom
C117  DNP/0.5pF  [C0402]  74.6,102.64 90 bottom
C118  18pF  [C0402]  61.6,100.71 0 bottom
C119  33nF  [C0402]  67.41,100.19 180 bottom
C120  1uF  [C0402]  67.44,99.3 180 bottom
C122  DNP/4.7uF  [C0805]  43,64.62 90 bottom
C124  DNP/18pF  [C0402]  79.83,66.88 90 bottom
C125  DNP/18pF  [C0402]  78.94,66.88 90 bottom
C126  39pF  [C0402]  57.61,64.54 90 bottom
C127  100nF  [C0402]  56.72,64.54 90 bottom
C128  22uF  [C0805]  59.13,63.75 90 bottom
C129  39pF  [C0402]  55.63,64.54 270 bottom
C130  39pF  [C0402]  53.54,64.54 270 bottom
C131  220pF  [C0402]  54.61,64.54 270 bottom
C132  1pF  [C0402]  43.03,70.59 90 bottom
C133  2.7pF  [C0402]  42.98,68.5 270 bottom
C134  2.2pF  [C0402]  49.91,67.14 270 bottom
C135  2.2pF  [C0402]  49.91,69.25 90 bottom
C136  1.5nF  [C0402]  51.44,70.24 0 bottom
C137  18pF  [C0402]  74.3,78.31 0 bottom
C138  18pF  [C0402]  69.57,78.82 0 bottom
C139  1uF  [C0402]  69.57,77.04 180 bottom
C140  10pF  [C0402]  69.57,77.93 180 bottom
C141  DNP/18pF  [C0402]  64.59,78.16 270 bottom
C142  1.2pF  [C0402]  61.9,78.16 270 bottom
C143  18pF  [C0402]  74.3,79.3 180 bottom
C144  18pF  [C0402]  74.3,77.32 180 bottom
C145  18pF  [C0402]  71.04,76.43 270 bottom
C148  DNP/EECENOF204Rk  [2P-D6.8MMX1.8MMH]  7.98,91.77 270 top
C151  4.7uF  [C0805]  51.74,80.01 90 top
C152  4.7uF  [C0805]  57.43,77.27 90 top
C153  22uF  [C0805]  14.11,66.5 90 top
C154  22uF  [C0805]  12.19,61.85 180 bottom
C155  22uF  [C0805]  12.19,63.88 180 bottom
C156  SMD CAP Tantalum 47uF-10V;B  [AVX-B]  12.7,66.42 180 bottom
C157  4.7nF  [C0402]  14.1,68.64 0 top
C158  33nF  [C0402]  22.35,69.72 180 top
D1  SS0520-7-F  [SOD123]  16.59,86.59 180 top
D2  MMSZ4689-V  [SOD123-2.7X1.6]  17.53,66.42 0 bottom
D3  CESD5V0AP  [SOT23]  18.24,97.89 180 top
D4  CESD5V0AP  [SOT23]  15.11,97.92 180 top
D6  CESD5V0AP  [SOT23]  11.25,83.03 270 top
D7  SS14  [D2010]  20.45,64.01 180 top
D15  SS0520-7-F  [SOD123]  31.22,62.86 180 bottom
DN  USB_DP  [TP_4545]  6.6,82.04 0 top
DP  USB_DN  [TP_4545]  6.6,83.95 0 top
GPS  U-FL Connector  [4P-U-FL]  80.09,101.3 180 bottom
GSM  U-FL Connector  [4P-U-FL]  82.68,65.53 180 bottom
J1  SMD Grove;4P-2.0  [4P-SMD-2.0]  36.32,96.01 270 top
J2  JST  [JST-SMD-2.0-90D]  3.94,61.72 270 top
J4  TF+SIM-VSHO-21-3301  [16P-L17.4MM*W16.5MM*H2.7MM]  10.29,85.85 90 bottom
J7  Micro USB 5P without POST;ST-USB-001G  [MICRO-USB]  4.7,82.68 270 top
J11  SMD Grove;4P-2.0  [4P-SMD-2.0]  45.85,96.01 270 top
J16  344017001  [8P-3.5-SMD]  -0.38,101.09 0 top
JTAG  DNP  [2*5P-2.0-TESTPOINT]  16.64,99.82 180 bottom
L  GREEN  [LED-0603]  23.62,96.19 0 top
L1  4.3nH  [L0402]  51.44,68.81 0 bottom
L2  Bead 120R-2A  [L0603]  51.26,77.44 0 top
L3  LQM2MPN2R2MG0  [0806]  59.74,90.98 270 bottom
L4  4.3nH  [L0402]  43.7,78.02 90 bottom
L5  6.8nH  [L0402]  65.53,101.73 0 bottom
L6  LQM2MPN2R2MG0  [0806]  51.51,76.45 180 bottom
L7  1.5nH  [L0402]  63.25,78.61 0 bottom
L8  SMD Power Inductor 10uH-20%;021042001  [L0630]  26.92,65.41 270 top
L9  BLM15BD182SN1  [L0402]  18.19,88.7 0 top
L10  BLM15BD182SN1  [L0402]  15.14,88.82 180 top
L11  100nH  [L0603]  12.6,94.08 180 top
L12  1nH  [L0402]  42.24,76.56 180 bottom
L13  SMD Power Inductor 10uH-20%;021042001  [L0630]  21.41,75.21 90 top
L14  1.8nH  [L0402]  44.15,76.56 180 bottom
L15  4.7nH  [L0402]  44.59,79.79 270 bottom
L16  4.3nH  [L0402]  51.44,67.59 0 bottom
L17  4.3nH  [L0402]  41.61,70.15 0 bottom
L18  3.3nH  [L0402]  59.23,102.06 90 bottom
L19  4.3nH  [L0402]  41.55,68.96 0 bottom
L20  22nH  [L0603]  70.87,99.44 0 bottom
L21  BLM18BD252SN1  [L0603]  16.64,101.35 90 top
L22  BLM18BD252SN1  [L0603]  18.85,101.37 90 top
L23  BLM18BD252SN1  [L0603]  14.61,101.37 90 top
L24  470R-1000mA  [L0805]  12.2,66.5 90 top
P1  [ROUND-MARK-1.0]  1.68,107.67 0 top
P2  [ROUND-MARK-1.0]  80.19,58.7 0 top
P3  [ROUND-MARK-1.0]  1.68,107.67 0 bottom
P4  [ROUND-MARK-1.0]  80.19,58.7 0 bottom
P5  [ROUND-MARK-1.0]  not placed on the board
P6  [ROUND-MARK-1.0]  not placed on the board
P7  [ROUND-MARK-1.0]  not placed on the board
P8  [ROUND-MARK-1.0]  not placed on the board
P9  [ROUND-MARK-1.0]  not placed on the board
P10  [ROUND-MARK-1.0]  not placed on the board
P11  [ROUND-MARK-1.0]  not placed on the board
P12  [ROUND-MARK-1.0]  not placed on the board
PWR  GREEN  [LED-0603]  14.1,57.91 270 top
Q1  CJ2302  [SOT23]  7.75,61.09 270 bottom
Q2  CJ2302  [SOT23]  23.62,99.19 180 top
Q3  CJ2302  [SOT23]  29.34,91.59 270 bottom
Q4  CJ2302  [SOT23]  34.04,92.41 0 bottom
Q6  CJ2305  [SOT23]  29.97,99.19 180 top
Q7  CJ2305  [SOT23]  26.8,99.19 180 top
Q8  CJ2302  [SOT23]  37.34,99.11 0 bottom
Q9  CJ2302  [SOT23]  37.34,102.54 0 bottom
Q10  CJ2302  [SOT23]  37.34,95.55 0 bottom
Q11  CJ2302  [SOT23]  40.64,90.81 0 bottom
Q12  CJ2302  [SOT23]  40.64,102.54 0 bottom
Q13  CJ2302  [SOT23]  40.64,95.55 0 bottom
Q14  S8550  [SOT23]  3.3,64.26 270 bottom
R1  0R  [R0402]  60.43,69.06 180 bottom
R2  10K  [R0402]  21.74,84.56 0 bottom
R3  100K  [R0402]  54.43,76.53 270 bottom
R4  49.9R-1%  [R0402]  55.91,78.05 270 top
R5  910K  [R0402]  56.34,83.74 180 top
R6  10K  [R0402]  50.27,82.3 0 bottom
R7  1K  [R0402]  10.57,86.49 180 top
R8  1.5K  [R0402]  22.1,85.09 0 top
R10  100R  [R0402]  18.24,93.4 0 top
R11  100R  [R0402]  15.14,93.4 0 top
R12  1K  [R0402]  32.74,73.1 0 top
R13  1.5K  [R0402]  27.03,74.8 270 bottom
R14  1.5K  [R0402]  27.51,76.45 180 bottom
R15  470R  [R0402]  15.14,95.43 180 top
R16  470R  [R0402]  18.24,95.43 180 top
R17  0R  [R0402]  8.51,83.64 0 top
R18  0R  [R0402]  8.51,82.45 0 top
R19  10K  [R0402]  28.78,82.68 180 bottom
R20  10K  [R0402]  29.11,85.24 0 bottom
R21  0R  [R0402]  79.38,83.31 0 bottom
R22  0R  [R0402]  34.54,100.56 180 top
R23  0R  [R0402]  34.49,101.6 180 top
R24  10K  [R0402]  36.22,80.72 180 top
R25  0R  [R0402]  13.08,95.4 180 top
R26  DNP/0R  [R0402]  49.89,98.37 180 bottom
R27  0R  [R0402]  33.48,97.16 180 top
R28  0R  [R0402]  33.48,98.17 180 top
R29  100K  [R0402]  25.3,101.98 270 top
R30  3.9k  [R0402]  16.38,68.58 0 top
R31  DNP/0R  [R0402]  49.89,97.49 180 bottom
R32  0R  [R0402]  50.27,81.31 0 bottom
R33  10K  [R0402]  14.99,73.23 90 top
R34  33K-1%  [R0402]  12.52,72.76 0 top
R35  8.2K-1%  [R0402]  11,75.22 90 top
R36  1K  [R0402]  21.26,60.07 90 bottom
R37  DNP/10K  [R0402]  33.86,80.72 0 top
R38  0R  [R0402]  19.53,95.22 0 bottom
R39  100R  [R0402]  19.53,101.88 0 bottom
R40  1K  [R0402]  4.06,107.06 180 top
R41  0R  [R0402]  65.53,100.2 180 bottom
R45  33K-1%  [R0402]  43.03,62.31 0 bottom
R46  4.7K  [R0402]  39.5,98.93 90 bottom
R47  100R  [R0402]  18.21,60.07 270 bottom
R48  10R  [R0402]  14.22,78.46 90 top
R49  1K  [R0402]  22.73,101.98 90 top
R50  33K-1%  [R0402]  12.52,74.78 180 top
R51  0R  [R0402]  12.52,73.76 0 top
R52  0R  [R0402]  56.52,101.47 270 bottom
R53  47K  [R0402]  5.97,107.06 0 top
R54  0R  [R0402]  79.38,65.53 0 bottom
R55  0R  [R0402]  52.53,64.54 270 bottom
R56  24K  [R0402]  54.56,62.64 270 bottom
R57  10K  [R0402]  53.54,62.64 270 bottom
R58  33K-1%  [R0402]  48.51,63.63 180 bottom
R59  33K-1%  [R0402]  45.14,63.83 90 top
R60  0R  [R0402]  55.63,62.64 270 bottom
R61  0R  [R0402]  63.25,77.72 0 bottom
R62  68k  [R0402]  16.38,66.8 0 top
R63  100R  [R0402]  19.53,100.89 0 bottom
R64  100R  [R0402]  19.53,96.27 0 bottom
R65  100R  [R0402]  19.53,97.28 0 bottom
R66  100R  [R0402]  19.53,98.3 0 bottom
R67  DNP/1K  [R0402]  40.01,76.81 90 top
R68  100R  [R0402]  19.53,99.87 180 bottom
R69  10K  [R0402]  33.02,99.69 90 bottom
R70  330K  [R0402]  7.75,58.29 270 bottom
R71  4.7K  [R0402]  29.34,94.28 180 bottom
R72  10K  [R0402]  21.89,87.5 180 bottom
R73  4.7K  [R0402]  32.51,94.23 0 bottom
R74  10K  [R0402]  21.74,83.49 0 bottom
R75  10K  [R0402]  51.51,64.54 270 bottom
R76  1K  [R0402]  29.16,101.98 90 top
R77  1K  [R0402]  26.19,101.98 90 top
R78  1K  [R0402]  12.7,58.42 90 top
R79  0R  [R0402]  75.06,101.3 0 bottom
R80  DNP/0R  [R0402]  53.01,101.47 270 bottom
R81  1K  [R0402]  20.24,60.07 90 bottom
R82  4.7K  [R0402]  35.26,102.39 270 bottom
R83  4.7K  [R0402]  35.26,99.09 270 bottom
R84  10K  [R0402]  34.62,74.07 180 top
R85  10K  [R0402]  39.98,78.59 270 top
R86  39K  [R0402]  8.79,58.29 90 bottom
R87  10K  [R0402]  60.15,83.62 0 top
R88  33K-1%  [R0402]  45.14,61.9 270 top
R89  33K-1%  [R0402]  46.25,61.9 270 top
R90  33K-1%  [R0402]  47.37,61.9 270 top
R91  24k  [R0402]  16.38,67.69 0 top
R92  10K  [R0402]  60.15,84.51 0 top
R93  3.3K  [R0402]  6.98,63.63 180 bottom
R94  0.2R-0805-1%  [R0805]  7.75,65.53 0 bottom
R96  10K  [R0402]  35.2,78.59 270 top
R97  10K  [R0402]  34.26,78.59 270 top
R98  4.7K  [R0402]  31.88,91.64 270 bottom
R99  4.7K  [R0402]  36.96,91.57 180 bottom
R104  DNP/0R  [R0402]  35.99,70.48 270 bottom
R105  100R  [R0402]  34.62,73.1 180 top
R106  1K  [R0402]  30.86,101.98 90 top
R107  1K  [R0402]  27.69,101.98 90 top
R108  10K  [R0402]  24.41,101.98 270 top
R109  10K  [R0402]  49.89,96.6 180 bottom
R110  DNP/10K  [R0402]  53.9,101.47 270 bottom
R111  4.7K  [R0402]  34.06,102.44 270 bottom
R112  4.7K  [R0402]  36.96,93.14 0 bottom
R113  4.7K  [R0402]  35.1,95.5 270 bottom
R114  4.7K  [R0402]  40.64,88.39 0 bottom
R115  4.7K  [R0402]  41.5,98.98 270 bottom
R116  4.7K  [R0402]  44.88,102.57 270 bottom
R117  4.7K  [R0402]  42.8,102.54 270 bottom
R118  4.7K  [R0402]  40.64,93.14 0 bottom
R119  4.7K  [R0402]  43.87,102.54 270 bottom
RESET  SMD Button;TS-1188E 6C81  [4P-SMD-7X3.5X3.5H]  19.81,58.04 0 top
RST  RED  [LED-0603]  25.53,57.91 270 top
RX  RED  [LED-0603]  29.97,96.19 0 top
SW1  [3P-SMD-2CH-6.6X2.8-REINFORCE]  26.67,84.2 0 top
SW2  [3P-SMD-2CH-6.6X2.8-REINFORCE]  2.01,71.88 0 top
SW3  SWITCH-2CH-6P-2.54  [6P-2CH-2.54-7.6X3.0]  7.75,71.88 180 top
TX  RED  [LED-0603]  26.8,96.16 0 top
U1  MT5931  [TFBGA84]  56.01,82.3 180 bottom
U2  MT3332  [QFN48-6X6MM]  54.74,96.77 270 bottom
U3  MX25U12835FZNI10G  [WSON8-6X5X0.8H-W/HEAT]  35.69,83.85 270 bottom
U4  XC6221B332MR-G  [SOT-25J]  55.58,90.17 270 top
U6  BCT4699  [TQFN16]  29.34,92.2 0 top
U7  MT2502A  [VFBGA143]  35.94,76.33 90 bottom
U8  NC/STT818B  [SOT23-6L]  3.3,60.45 180 bottom
U9  EPCOS LZ97A  [5P-SMD-1.4X1.1MM]  69.32,101.3 0 bottom
U10  [SHIELD-SMD-44.5X53.5]  23.62,104.9 180 bottom
U11  PCB  [ARDUINO-38P]  0.13,56.01 0 top
U12  MP1496  [TSOT23-8]  15.52,75.9 90 top
U13  MAX2659  [6P-SMD-1.5X1.0X0.72H]  63.55,101.22 180 bottom
U14  RF7198  [32P-SMD-RF1798-5.3MMX5.25MMX0.73H]  56.01,68.71 180 bottom
U15  FB2012-05N2R4GT  [8P-SMD-2X1.25X0.7H]  66.83,78.16 90 bottom
U16  uPG2176T5N  [TSON6]  71.88,78.31 0 bottom
U17  DNP/BAV70S  [SOT363]  45.57,63.14 90 bottom
U18  TXS0108PW  [TSSOP20]  28.6,99.16 0 bottom
U19  CJA1117B-3.3  [SOT89]  46.02,94.61 0 bottom
U20  ISL97516  [MSOP8]  20.45,67.44 270 top
U$13  [OSHW_FILLX200_NOTEXT]  74.42,66.17 90 top
U$14  [MTK-LINKLTONE]  30,81.94 0 top
U$15  [BYMTK-200-1]  74.42,79.5 90 top
U$18  [LOGO_SILK]  72.52,75.69 90 top
VBAT_TP  VBAT  [TP_4545]  14.71,63.63 0 bottom
VCHG_5V1  [TP_4545]  14.73,61.09 0 bottom
VIO_28  [TP_4545]  17.27,63.63 0 bottom
WI-FI/BT  U-FL Connector  [4P-U-FL]  82.68,83.31 180 bottom
X1  SMD Crystal 32.768KHZ-12.5pF-20ppm-80K  [2P-SMD-2.05X1.2]  29.51,78.33 270 bottom
X2  7L26002009  [2520]  63.63,96.65 90 bottom
X3  7M26000028/TXC  [4P-SMD-3.2X2.5]  43.18,73.61 0 bottom

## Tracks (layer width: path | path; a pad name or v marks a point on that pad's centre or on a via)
2G_ANT
  Bottom 0.132: U14.19 59.91,68.99 R1.1 59.97,69.08 C82.1
2G_XTAL1
  Bottom 0.102: 38.16,75.13 38.21,75.13 38.28,75.06 38.63,75.06 40.31,73.38 43.51,73.38 44.27,72.62
  Bottom 0.132: U7.B4 38.16,75.13
  Bottom 0.152: X3.1 44.3,72.59 44.27,72.62
2G_XTAL2
  Bottom 0.102: X3.3 41.91,73.86 41.63,73.58 40.36,73.58 38.68,75.26 38.41,75.26 U7.B5
  Bottom 0.132: U7.B5
5V_OUT  (via drill 0.3 pad 0.51)
  Top 0.61: J1.3 36.14,95.01 34.01,95.01 C28.1 C90.1 | 42.42,95.01 41.28,95.01 | v43.43,93.34 43.43,94.49 | 43.43,94.49 43.43,94.5 42.93,95.01 | 43.43,94.49 43.94,95 | v47.68,81 47.68,79.02 49.51,77.19 49.51,67.23 50.93,65.81 51.44,65.81 v51.49,65.86
  Top 0.813: J11.3 42.93,95.01 42.42,95.01 41.54,95.01 | 41.54,95.01 41.28,95.01 | 41.54,95.01 41.53,95.02 36.15,95.02 36.14,95.01
  Top 1.016: v11.23,67.69 11.53,67.39 L24.2
  GND 0.406: v11.3,60.58 11.43,60.58 11.56,60.45
  GND 0.61: v51.49,65.86 51.49,65.81 49.55,63.88 42.19,63.88 v41.58,64.49
  GND 1.016: v20.07,61.98 18.54,60.45 11.56,60.45 11.3,60.45
  Bottom 0.61: v43.43,93.34 43.56,93.34 43.82,93.09 44.45,93.09 44.45,92.91 44.37,92.84 U19.3 44.5,91.9 45.47,90.93 C1.1 45.33,90.64 C108.1 45.33,88.53 47.12,86.74 47.12,84.45 47.88,83.69 47.88,81.2 v47.68,81 | U11.28 36.83,59.94 36.83,64.11 37.21,64.49
  Bottom 1.016: v41.58,64.49 37.21,64.49 34.82,64.49 33.78,65.53 23.62,65.53 v20.07,61.98 | v11.3,60.58 C154.1 C155.1 11.3,66.36 C156.+ 11.24,67.68 v11.23,67.69
/M_SCL  (via drill 0.1 pad 0.25 layers 15-16, 0.2 pad 0.41 layers 2-15, 0.3 pad 0.51)
  GND 0.152: v37.31,90.6 38.58,89.33 38.58,82.37 39.01,81.94 v39.01,81.74
  GND1 0.076: U7.B11 38.14,78.38 38.38,78.61 38.88,78.61 39.26,78.99 39.26,80.15 39.42,80.31 39.42,81.33 v39.01,81.74
  Bottom 0.152: R99.2 37.31,91.48 v37.31,90.6 37.26,90.55 33.98,90.55 Q4.2
  other vias: 38.14,77.93
/M_SDA  (via drill 0.1 pad 0.25 layers 15-16, 0.2 pad 0.41 layers 2-15, 0.3 pad 0.51)
  Top 0.152: 44.2,87.07 37.59,87.07 36.8,86.28 35.28,86.28 31.93,89.64 31.93,89.99 31.42,90.5 v31.28,90.5 | 44.2,87.07 44.22,87.07 | 44.2,87.07 v44.37,87.25
  GND 0.102: v38.04,76.38 38.76,76.38 39.62,77.24 40.01,77.62 40.01,78.77 39.65,79.12 39.65,79.53 39.8,79.68 40.92,79.68
  GND 0.152: 40.92,79.68 42.29,81.05 42.29,85.17 v44.37,87.25
  GND1 0.152: v37.74,76.32 37.98,76.32 v38.04,76.38
  Bottom 0.152: U7.C7 v37.74,76.32 | R98.2 31.88,91.1 v31.28,90.5 30.56,90.5 Q3.2
/SPI_MISO  (via drill 0.3 pad 0.51)
  Top 0.152: U6.7 29.59,90.09 29.29,89.79 v29.18,89.79
  Bottom 0.152: v29.18,89.79 28.02,89.79 27.2,90.6 27.2,94.16 26.85,94.51 26.85,95.38 26.95,95.48 26.95,96.07 U18.8
/SPI_MOSI  (via drill 0.3 pad 0.51)
  Top 0.152: v27.36,94.97 27.91,94.41 28.97,94.41 29.08,94.3 U6.15
  Bottom 0.152: U18.7 27.62,95.24 v27.36,94.97
/SPI_SCL  (via drill 0.3 pad 0.51)
  Top 0.152: U6.3 26.93,91.95 v26.59,91.62 | v26.34,94.97 25.58,94.97 25.22,95.33 25.22,98.05 23.74,99.53 23.74,101.77 24.26,102.29 24.27,102.29 R108.1
  Bottom 0.152: v26.59,91.62 26.91,91.93 26.91,93.95 26.34,94.51 v26.34,94.97 26.34,96.08 U18.9
/SPI_SS  (via drill 0.3 pad 0.51)
  Top 0.152: v29.97,89.79 29.97,89.1 34.07,85.01 37.46,85.01 38.33,85.88 45.72,85.88 v46,86.16
  GND 0.152: v44.15,82.3 44.15,82.45 44.53,82.83 45.84,82.83 47.03,84.01 47.03,85.05 46,86.08 v46,86.16
  Bottom 0.076: 28.27,95.83 U18.6
  Bottom 0.102: U7.B13 38.99,79.58 41.98,79.58 42.9,80.49 42.9,80.75 | 43,82.02 43.31,82.32
  Bottom 0.152: 42.9,80.75 42.9,81.91 43.31,82.32 44.12,82.32 v44.15,82.3 | v29.97,89.79 29.9,89.79 29.44,90.25 28,90.25 27.51,90.74 27.51,94.21 27.86,94.56 27.86,95.07 28.27,95.48 28.27,95.83
ACCDET  (via drill 0.1 pad 0.25 layers 15-16, 0.2 pad 0.41 layers 2-15, 0.3 pad 0.51)
  GND 0.152: v33.15,74.91 33.06,74.82 31.58,74.82 31.27,74.5 30.5,74.5 28.93,76.07 v28.22,76.07
  GND1 0.076: v33.15,74.91 33.94,74.91 34.56,75.53 U7.K5
  GND1 0.102: U7.K5 34.89,75.53
  Bottom 0.152: R14.2 27.96,76.44 27.96,76.33 v28.22,76.07
  other vias: 34.94,75.53
AD0/D14
  Top 0.152: 45.12,61.45 R88.2 46.01,60.58 46.05,60.58 46.36,60.58 47.37,60.58 47.68,60.27 49.2,60.27 U11.19
AD1/D15
  Top 0.152: 46.24,61.45 R89.2 46.83,60.88 47.47,60.88 47.78,60.58 51.44,60.58 U11.20
AD2/D16
  Top 0.152: U11.21 53.67,60.88 47.94,60.88 R90.2
ANTSEL_0
  Bottom 0.152: U16.1 73.36,78.81 C143.1 73.85,84.95 70.14,88.66 60.28,88.66 57.1,85.47 57.1,84.7 U1.K8
ANTSEL_1  (via drill 0.3 pad 0.51)
  GND 0.152: v73.2,79.86 74.57,78.49 v74.57,76.43
  Bottom 0.076: U1.J8 57.51,84.3 57.51,84.71 57.4,84.81
  Bottom 0.152: U16.3 73.36,77.81 C144.1 73.81,77.28 73.81,76.68 74.07,76.43 v74.57,76.43 | 57.4,84.81 57.4,85.34 60.39,88.33 70.04,88.33 73.2,85.17 v73.2,79.86
APC_VBAIS  (via drill 0.1 pad 0.25 layers 15-16, 0.2 pad 0.41 layers 2-15, 0.3 pad 0.51)
  GND 0.203: v52.76,62.81 52.76,66.87 51.88,67.74 41.48,67.74 37.72,71.5 32.69,71.5 32.39,71.5 32.13,71.5 v32.11,71.53
  GND1 0.152: v32,76.33 31.37,76.33 31,75.96 31,72.63 v32.11,71.53
  Bottom 0.102: U7.N7 v32,76.33
  Bottom 0.152: R57.2
  Bottom 0.203: 53.33,62.19 R57.2 53.07,62.19 52.76,62.51 v52.76,62.81
AUDIO_GND  (via drill 0.3 pad 0.51)
  Top 0.305: 14.22,98.68 D4.2 14.35,99.06 14.35,99.09 12.64,97.37 v12.64,96.14 12.64,95.73 R25.2 12.61,95.38 | J16.2 5.32,97.6 | 5.41,97.55 J16.2 | J16.2 5.32,97.09 v6.17,96.24
  GND 0.305: v6.17,96.24 12.54,96.24 v12.64,96.14
AVDD_SMPS  (via drill 0.3 pad 0.51)
  Top 0.152: 54.48,78.16 C12.1
  Top 0.305: 54.48,78.16 v54.48,78.92
  Top 0.406: v52.6,78.92 52.1,78.92 51.89,79.12
  Top 0.61: C151.1 51.89,79.12 51.99,79.12 52.05,79.07 52.05,77.47 L2.2 53.52,77.44 54.13,78.05 54.38,78.05 C12.1
  Bottom 0.076: U1.A4 55.23,80.05 | 54.27,80.03 U1.A2
  Bottom 0.152: U1.A2 54.26,80.01
  Bottom 0.254: U1.A4 55.26,79.69 v54.48,78.92 | v52.6,78.92 53.11,78.92 54.24,80.05 U1.A2
BANDSW  (via drill 0.1 pad 0.25 layers 1-2, 0.1 pad 0.25 layers 15-16, 0.2 pad 0.41 layers 2-15, 0.3 pad 0.51)
  Top 0.152: v51.44,63.32 51.03,63.73 50.52,63.73 47.27,66.98 47.27,73.38 45.75,74.91 45.75,78.33 v45.8,78.38
  GND 0.102: v45.8,78.38 45.62,78.21 42.25,78.21 41.15,77.1 41.15,76.19 40.65,75.69 40.01,75.69 v39.79,75.47
  GND1 0.076: U7.D5 37.45,75.64 39.63,75.64 v39.79,75.47
  GND1 0.102: U7.D5 37.35,75.53
  Bottom 0.152: R60.2 55.63,62.03 54.88,61.28 53.02,61.28 51.44,62.86 v51.44,63.32
  other vias: 37.34,75.53
BAT_CHARGE
  Bottom 2.032: R94.1 8.64,66.93 SW3.CH2A
  pour Bottom (isolate 0.254, no thermals): 8,64.9 9.27,64.9 9.27,66.55 8,66.55
BATON  (via drill 0.1 pad 0.25 layers 1-2, 0.1 pad 0.25 layers 15-16, 0.2 pad 0.41 layers 2-15)
  Top 0.102: 35.08,74.05 R84.1
  Top 0.152: 35.08,74.05 35.52,74.05 v35.54,74.04
  GND 0.152: v35.54,74.04 35.59,74.04 v35.94,74.4
  GND1 0.102: v35.74,75.51 35.74,75.23 35.94,75.03 v35.94,74.4
  Bottom 0.102: U7.H5 v35.74,75.52 v35.74,75.51
BATTERY
  Top 0.254: 8.13,63.37 8.37,63.37 J2.+ 9.02,63.5
  Top 2.032: SW3.CH1A 8.38,68.45 8.38,63.39 8.37,63.37
  pour Top (isolate 0.254, no thermals): 7.24,62.61 7.24,64.01 arc-90 7.49,64.26 10.54,64.26 arc-90 10.79,64.01 10.79,62.61 arc-90 10.54,62.36 7.49,62.36 arc-90
BPI_BUS2  (via drill 0.3 pad 0.51)
  Top 0.406: R67.2 40.01,78 40.01,78.09 40.01,78.12 R85.2 39.82,78.14 v39.4,78.56
  Bottom 0.203: U7.A12 38.65,78.33 38.89,78.56 v39.4,78.56
BT_ANT
  Bottom 0.132: C111.1 L14.2 C110.1 46.04,76.56 arc-45 46.45,76.39 47.85,74.98 arc45 48.16,74.85 70.11,74.85 arc90 71.04,75.79 C145.2
BT_LNA
  Bottom 0.102: U7.A6 38.58,75.93
  Bottom 0.132: 41.77,76.53 L12.1 | L12.1 C114.1 | U7.A6 40.6,75.93 arc45 40.99,76.09 41.21,76.31 arc-45 L12.1
BUCK_VBAT
  Top 0.152: C78.2 13.01,72.8 R34.2
  Top 0.203: C78.2 14.08,71.59 C79.1
  Top 1.27: SW3.CH2B SW3.CH1B 10.79,72.9 10.79,72.25 11.74,71.3 C79.1 14.38,70.33 14.48,70.23 14.93,69.78 18.85,69.78 21.34,72.26 21.34,72.28 L13.1
CHR_LDO  (via drill 0.1 pad 0.25 layers 15-16, 0.3 pad 0.51)
  GND 0.152: v31.9,69.42 31.9,68.68 33,67.59 v33,67.13 | 9.65,61.59 v9.53,61.72 9.73,61.52 17.45,61.52 v17.65,61.72
  GND1 0.102: v33.5,72.31 34.07,72.31 35.54,73.78 35.54,74.52 35.64,74.62 v35.64,74.91
  Bottom 0.102: 36.11,75.48 36.11,75.53 U7.G5 36.14,75.51 35.64,75.01 v35.64,74.91
  Bottom 0.152: v33.5,72.31 33.5,71.6 31.9,70 v31.9,69.42 | v33,67.13 33,67.08 32.54,66.62 23.24,66.62 18.85,62.23 18.16,62.23 v17.65,61.72 | v9.53,61.72 9.02,61.72 Q1.1 8.57,62.17 C48.1 R93.2
CLDO  (via drill 0.3 pad 0.51)
  Top 0.152: 55.72,82.89 55.72,82.97 v55.65,83.03
  Top 0.305: C21.1 55.97,82.72 v55.65,83.03 55.23,83.45 54.49,83.45 54,82.96 C22.1 | v52.98,81.05 52.98,82.07 53.75,82.83 C22.1 | 53.98,82.8 C22.1
  Bottom 0.152: U1.G7 U1.G6 56.24,83.03 v55.65,83.03 55.27,83.03 U1.G4
  Bottom 0.254: U1.G4 56.73,83.05 56.74,83.03
  Bottom 0.305: U1.C1 v52.99,81.05 v52.98,81.05
CMCSD0  (via drill 0.3 pad 0.51)
  Top 0.152: U6.4 27.66,91.28 27.66,89.64 28.02,89.28 29.39,89.28 33.95,84.72 37.58,84.72 38.43,85.57 47.75,85.57 v47.9,85.72
  GND 0.152: v43.66,81.86 43.94,81.86 44.32,81.48 44.32,81.2 44.43,81.1 44.58,81.1 44.68,81.2 44.68,81.76 44.78,81.86 44.93,81.86 45.03,81.76 45.03,80.75 45.14,80.64 45.29,80.64 45.39,80.75 45.39,81.93 45.68,82.22 46.56,82.22 46.8,82.46 46.98,82.46 47.6,81.84 47.75,81.84 47.85,81.94 47.85,82.09 47.22,82.73 47.22,82.88 47.32,82.98 47.47,82.98 47.49,82.97 | 48,83.47 47.98,83.49 47.83,83.49 47.73,83.39 47.73,83.24 48.36,82.6 48.36,82.45 48.26,82.35 48.11,82.35 47.49,82.97 | 47.49,82.97 47.3,82.97 | 47.81,83.47 48,83.47 | 48,83.47 48.62,82.85 48.77,82.85 48.87,82.96 48.87,83.11 48.06,83.92 48.06,84.08 48.13,84.15 48.77,84.15 48.87,84.25 48.87,84.4 48.77,84.51 47.99,84.51 47.89,84.61 47.89,84.76 47.99,84.86 48.77,84.86 48.87,84.96 48.87,85.11 48.77,85.22 48.03,85.22 47.9,85.34 v47.9,85.72
  Bottom 0.102: U7.A13 39.19,79.38 42.05,79.38 43.21,80.53 43.21,80.75
  Bottom 0.152: 43.21,80.75 43.21,81.71 43.36,81.86 v43.66,81.86
CMCSD1  (via drill 0.1 pad 0.25 layers 15-16, 0.2 pad 0.41 layers 2-15, 0.3 pad 0.51)
  Top 0.152: U6.16 26.19,93.7 25.92,93.44 25.92,90.91 27.86,88.98 29.29,88.98 33.84,84.42 37.68,84.42 38.53,85.27 48.13,85.27 v48.57,85.7
  GND 0.076: v39.29,75.31 39.48,75.12 39.92,75.12 40.31,75.51 40.72,75.51 41.33,76.12 41.33,76.99 42.29,77.95 42.49,77.95
  GND 0.152: 42.49,77.95 47.42,77.95 v47.57,78.1
  GND1 0.076: U7.E5 36.94,75.45 37.21,75.18 37.39,75.18 37.67,75.46 39.14,75.46 v39.29,75.31
  GND1 0.102: U7.E5
  Bottom 0.152: v47.57,78.1 47.57,79.32 48.43,80.17 48.43,85.56 v48.57,85.7
  other vias: 36.94,75.53
CMMCLK  (via drill 0.1 pad 0.25 layers 15-16, 0.2 pad 0.41 layers 2-15, 0.3 pad 0.51)
  Top 0.152: U6.8 30.09,90.41 30.45,90.04 30.45,89.59 30.61,89.43 30.61,89.33 30.45,89.18 30.45,89.03 30.56,88.92 30.71,88.92 30.84,89.05 30.99,89.05 31.09,88.95 31.09,88.8 30.96,88.67 30.96,88.52 31.06,88.42 31.22,88.42 31.5,88.7 31.65,88.7 31.75,88.59 31.75,88.44 31.47,88.16 31.47,88.01 31.57,87.91 31.72,87.91 32,88.19 32.16,88.19 32.26,88.09 32.26,87.94 31.98,87.66 31.98,87.5 32.08,87.4 32.23,87.4 32.51,87.68 32.66,87.68 32.77,87.58 32.77,87.43 32.49,87.15 32.49,87 32.59,86.89 32.74,86.89 33.02,87.17 33.17,87.17 33.27,87.07 33.27,86.92 33,86.64 33,86.49 33.1,86.38 33.25,86.38 33.53,86.66 33.68,86.66 33.78,86.56 33.78,86.41 33.5,86.13 33.5,85.98 33.6,85.88 33.76,85.88 34.04,86.16 34.19,86.16 34.29,86.05 34.29,85.9 34.01,85.62 34.01,85.47 34.16,85.32 34.37,85.32 34.57,85.52 34.77,85.52 34.93,85.37 37.31,85.37 38.12,86.18 45.21,86.18 v45.36,86.33
  GND 0.152: v43.31,81 43.21,81.1 43.21,82.22 43.61,82.63 43.61,83.28 43.73,83.39 44.07,83.39 44.17,83.49 44.17,83.64 44.07,83.74 43.66,83.74 43.56,83.84 43.56,84.05 43.66,84.15 44.37,84.15 45.09,83.44 45.24,83.44 45.37,83.57 45.37,83.71 44.22,84.86 44.22,85.01 44.32,85.11 44.48,85.11 45.94,83.66 46.09,83.66 46.19,83.76 46.19,83.91 44.78,85.32 44.78,85.47 44.88,85.57 45.03,85.57 46.44,84.16 46.6,84.16 46.7,84.27 46.7,84.41 45.36,85.75 v45.36,86.33
  GND1 0.102: v43.31,81 42.03,81 40.92,79.89 40.92,77.65 v40.41,77.14
  Bottom 0.076: U7.B9 38.17,77.13 38.32,77.28 arc-45 38.61,77.39 38.72,77.39
  Bottom 0.102: 38.72,77.39 40.16,77.39 v40.41,77.14
CMRST/EINT15  (via drill 0.1 pad 0.25 layers 15-16, 0.2 pad 0.41 layers 2-15, 0.3 pad 0.51)
  GND 0.152: v38.56,78.28 38.56,78.38 38.05,78.89 38.05,80.62 38.43,81 38.85,81 39.45,81.59 39.45,82.63 39.19,82.88 39.19,90.6 38.33,91.47 37.62,91.47 37.01,92.07 37.01,93.73 34.1,96.65 30.5,96.65 v29.95,97.21
  GND1 0.152: 38.53,77.78 v38.39,77.63
  GND1 0.254: v38.56,78.28 38.56,77.8 v38.39,77.63
  Bottom 0.152: U7.B10 38.28,77.53 v38.39,77.63 | U18.3 30.2,96.12 30.2,96.95 v29.95,97.21
D8/GPIO48/EINT21
  Bottom 0.152: U11.9 41.78,103.56 | Q12.3 41.78,103.56 | R117.1 42.23,103.56 42.14,103.56 41.78,103.56
DRV  (via drill 0.3 pad 0.51)
  GND 0.152: v32.56,69.42 32.56,68.68 33.71,67.54 v33.71,67.13 | v9.63,59.97 10.87,61.21 17.91,61.21 v18.41,61.72
  Bottom 0.102: U7.J2 35.34,74.3 35.23,74.19 35.23,73.48 33.76,72.01 33.76,71.45 33.6,71.3 32.66,70.36
  Bottom 0.152: v33.71,67.13 32.84,66.27 23.34,66.27 18.8,61.72 v18.41,61.72 | v9.63,59.97 8.99,59.97 Q1.2 | v32.56,69.42 32.56,70.26 33.6,71.3
EAR_EINT  (via drill 0.1 pad 0.25 layers 15-16, 0.2 pad 0.41 layers 2-15, 0.3 pad 0.51)
  Top 0.152: v46.91,81.05 46.91,80.9 47.07,80.75 47.07,77.06 v47.57,76.56
  Top 0.305: R40.1 4.51,107.61 v4.5,107.62
  GND 0.102: v41.05,74.35 41.05,74.57 41.22,74.75 41.22,75.01 42.04,75.82 42.04,76.48 42.29,76.73 42.49,76.73
  GND 0.152: 42.49,76.73 47.4,76.73 v47.57,76.56 | v4.5,107.62 7.39,107.62 10.24,104.78 18.92,104.78 20.24,103.45 20.24,100.56 20.6,100.2 21.97,100.2 22.68,99.49 31.67,99.49 32.89,98.27 34.57,98.27 38.12,94.72 38.49,94.72 39.55,93.66 39.55,93.65 42.6,90.6 42.6,90.32 43.07,89.84 43.97,89.84 v44.53,90.4
  GND1 0.076: U7.A3 38.68,74.73 39.01,74.4 39.35,74.4 39.64,74.1 40.22,74.1 40.28,74.17 40.87,74.17 v41.05,74.35
  GND1 0.102: U7.A3 38.54,74.71
  Bottom 0.152: v46.91,81.05 47.37,81.51 47.37,83.39 43.71,87.05 43.71,89.59 v44.53,90.4
  other vias: 38.54,74.73
EINT_WIFI  (via drill 0.1 pad 0.25 layers 1-2, 0.1 pad 0.25 layers 15-16, 0.2 pad 0.41 layers 2-15, 0.3 pad 0.51)
  Top 0.152: v51.28,82.17 50.65,82.17 50.29,82.53 45.64,82.53 44.48,81.36 41.35,81.36 v40.56,80.57
  GND 0.152: 40.54,80.54 v40.26,80.54 40.54,80.54 v40.56,80.57
  GND1 0.076: v40.26,80.54 40.26,79.83 40.51,79.58 40.51,77.92 39.32,76.73 39.11,76.73 38.8,76.41 38.47,76.41 38.18,76.7 v37.74,76.7
  Bottom 0.076: U1.E2 54,81.79 53.54,81.79 53.47,81.86 53.06,81.86
  Bottom 0.102: v37.74,76.7 U7.C8
  Bottom 0.152: U1.E2 | R6.1 51.16,82.3 v51.28,82.17 51.59,81.86 53.06,81.86 | v37.74,76.7 U7.C8 v37.74,76.71
FB_OUT
  Top 0.305: R62.1 C4.1 15.63,65.61 C153.1
  Top 1.016: D7.- 17.53,63.25 15.08,63.25 C88.+ 14.99,63.63 14.11,64.5 C153.1 L24.1
FM_ANT_P-1  (via drill 0.3 pad 0.51)
  Top 0.305: R25.1 13.51,95.39 13.51,94.23 L11.1
  Top 0.406: 13.59,93.85 13.54,93.9 | 13.54,93.9 L11.1 | 13.54,93.9 13.54,93.27 v13.59,93.22
  Bottom 0.102: U7.F2 36.54,74.3 36.66,74.19 36.66,73.2
  Bottom 0.152: 36.66,73.2 36.66,73.08 35.99,72.41 R104.1 | R104.1 | R104.1 35.46,70.4 35.46,69.49
  Bottom 0.305: v13.59,93.22 13.13,92.76 13.13,86.38 13.75,85.77 13.75,74.73 18.76,69.72 28.73,69.72 30.18,68.27 34.74,68.27 35.46,68.99 35.46,69.49
FREF_26M_WIFI  (via drill 0.3 pad 0.51)
  GND 0.152: v56.34,76.12 56.34,73.86 v56.39,73.81
  Bottom 0.132: 46.86,74.55 45.94,75.47 arc45 45.6,75.62 41.44,75.62 arc45 41.16,75.5 41.11,75.45 arc-45 40.65,75.26 39.54,75.26 arc-45 39.21,75.4 arc45 38.89,75.53 U7.A5
  Bottom 0.152: 46.86,74.55 47.46,73.95 arc45 47.86,73.79 56.36,73.79 v56.39,73.81 | v56.34,76.12 56.86,76.12 C20.1
GND  (via drill 0.1 pad 0.25 layers 1-2, 0.1 pad 0.25 layers 15-16, 0.2 pad 0.41 layers 2-15, 0.3 pad 0.51)
  Top 0.132: 56.83,82.49 56.86,82.49 56.87,82.47
  Top 0.152: v51.89,82.42 51.69,82.42 51.28,82.83 41.63,82.83 41.43,82.63 v41.43,81.99 | RX.- 30.73,96.11 30.15,95.53 28.83,95.53 | 28.83,95.53 28.19,95.53 TX.- | C87.2 28.89,95.47 28.83,95.53 | v29.59,74.6 C97.2 30.31,75.02 30.61,75.31 32.21,75.31 32.59,75.69 33.53,75.69 34.04,75.18 | v33.45,78.16 33.3,78 32.84,78 31.88,78.97 31.37,78.97 | C96.2 30.31,77.51 v30.61,77.8 | J1.4 36.32,91.62 35.76,91.06 31.11,91.06 30.76,90.7 30.76,89.74 31.17,89.33 31.42,89.33 35.08,85.67 37.16,85.67 37.97,86.49 44.73,86.49 45.03,86.79 46.66,86.79 47.22,86.23 48.84,86.23 49.05,86.03 49.05,84.96 | 49.05,84.96 38.99,84.96 37.97,83.95 v35.15,83.95 33.91,83.95 29.21,88.65 23.65,88.65 v23.37,88.37 | 49.05,84.96 50.29,84.96 50.62,85.29 53.11,85.29 v53.37,85.55 | 53.59,80.43 53.84,80.19 C14.1 | U6.6 29.09,91.37 v29.34,91.62 | 31.37,78.97 26.16,78.97 v22.68,82.45 21.49,83.64 13.74,83.64 12.52,84.86 | C9.2 arc45 36.22,78.13 37.01,78.92 arc45 37.18,78.99 37.26,79.07 | v53.26,66.17 53.21,66.17 52.32,65.28 50.67,65.28 48.77,67.18 48.77,74.85 v47.8,75.82 | R84.2 34.16,74.07 | v44.58,71.6 44.58,72.87 43.31,74.14 43.31,78.51 v43.26,78.56 | v46.08,79.65 46.15,79.58 46.15,75.06 47.57,73.63 47.57,67.1 50.44,64.24 50.93,64.24 | Q2.2 22.73,100.46 23.37,101.09 23.37,101.98 23.62,102.23 | C10.2 31.38,78.98 31.37,78.97 | v16.64,96.95 16.64,95.5 16.13,95 16.13,92.46 16.51,92.07 16.64,92.07 | 16.64,92.07 16.76,92.07 17.14,92.46 17.14,93.76 C54.2 | 16.64,92.07 16.64,89.79 | 16.64,89.79 v16.66,89.76 | 16.64,89.79 16.64,88.9 16.51,88.77 16.51,87.63
  Top 0.203: 30.3,77.39 29.84,77.85 25.63,77.85 21.11,82.37 13.69,82.37 11.96,80.64 5.97,80.64 5.24,81.38 J7.5 | v36.88,75.46 37.33,75.46 C71.2 | C151.2 52.05,80.9 52.05,81.2 | C23.2 55.63,85.19 54.89,85.93 51.38,85.93 51.33,85.98 | 51.23,77.95 51.23,76.58 51.28,76.53 | v55.27,82.12 55.04,82.12 54.99,82.17 53.66,82.17 53.47,81.98 53.47,80.56 53.84,80.19 | v55.73,75.31 55.73,76.4 56.06,76.73 57.28,76.73 57.84,76.17 57.84,75.31
  Top 0.254: v24.27,78.63 24.13,78.49 24.13,77.37 24.46,77.04 v24.84,77.04 | 57.94,80.95 v57.23,80.95
  Top 0.305: 54.58,89.97 U4.2 | C54.2 R16.2 17.79,96.28 18.26,96.75 18.26,96.85 D3.3 | R15.2 14.69,96.48 D4.3 | v53.57,76.28 53.59,76.3 54.27,76.3 C12.2 54.43,76.33 54.74,76.33 | 56.86,82.49 56.86,82.64 55.89,83.6 R5.2 | v50.81,80.58 51.42,80.58 C151.2 | C152.1 57.23,76.38
  Top 0.406: 22.53,86.96 C107.- | 30.86,96.32 RX.- 30.89,96.34 v30.89,97.87 | C90.2 C28.2 33.03,95.39 v33.02,95.4 | v38.1,93.32 37.59,93.32 37.16,92.89 36.45,92.89 J1.4 | 54.27,76.3 54.27,75.35 v54.23,75.31 | U11.35 67.82,81.41 | U11.35 65.02,81.41 | U11.35 66.17,80.26 | U11.35 66.17,82.55 | v43.16,92.63 44.63,92.63 44.98,92.99 45.82,92.99 J11.4
  Top 0.61: J1.4 36.32,93.12 36.3,93.14 | 45.82,93.04 J11.4
  GND 0.152: v41.89,82.6 41.89,85.47 44.12,87.71 44.48,87.71 47.83,91.06 49.68,91.06 v50.93,92.3 | v29.9,76.17 28.27,77.8 28.27,83.03 27.96,83.34 27.96,87.37 27.33,88.01 26.34,88.01 23.2,84.87 12.92,84.87 9.58,88.21 9.58,93.9 9.17,94.31 8.71,94.31 8.32,93.92 6.87,93.92 v6.43,94.36 | 19.63,86.08 13.48,86.08 12.5,87.06 12.5,87.07 10.79,88.77 10.79,92.69 11.66,93.55 | 19.63,86.08 22.58,86.08 25.73,89.23 27.91,89.23 29.18,87.96 29.18,83.95 29.49,83.64 29.49,78.51 30.2,77.8 v30.61,77.8 | v39.88,76.33 39.88,75.95 | 39.7,75.87 39.8,75.87 39.85,75.92 40.51,75.92 40.87,76.28 40.87,77.09 v40.69,77.27 | v38.94,74.3 38.94,74.35 | 40.72,78.46 44.7,78.46 v44.88,78.64 | v3.96,98.65 3.96,100.66 5.63,102.34 15.62,102.34 15.82,102.13 17.3,102.13 | 3.94,102.69 4.5,103.25 16.99,103.25 17.25,103 17.25,102.18 17.3,102.13 | v3.91,102.67 3.91,103.94 4.39,104.42 9.37,104.42 9.83,103.96 17.45,103.96 18.52,102.89 18.52,102.44 18.21,102.13 17.3,102.13 | 51,62.25 53.34,62.25 v55.12,64.03 | 19.63,86.08 19.63,86.44 20.55,87.35 20.55,89.33 23.98,92.76 v25.48,92.76 | 51,62.25 v50.75,62.51 | 41.43,82.02 41.38,82.07 41.33,82.07 41.21,82.19 41.21,85.66 43.87,88.32 44.02,88.32 48.08,92.38 49.12,92.38 v49.15,92.35 | v45.01,79.65 43.33,79.65 42.8,80.19 | 51,62.25 40.23,62.25 39.12,63.37
  GND 0.203: v42.04,75.16 41.73,75.16 41.48,74.91 41.48,73.74 | v46.08,79.65 47.4,79.65 48.23,80.49 48.23,81.86 49.33,82.96 49.33,83.46 49.25,83.54
  GND 0.254: v38.93,75.87 39.7,75.87
  GND 0.305: v33.45,76.68 33.45,77.29 33.2,77.55 33.2,77.9 33.33,78.03 | 33.33,78.03 v33.45,78.16 | v33.55,74.57 33.59,74.57 U7.K6 v35.25,75.93 v35.26,75.92 | v52.17,66.22 52.17,66.8 51.64,67.33 39.95,67.33 | 34.87,77.8 34.65,78.03 v33.83,78.03 33.33,78.03 | v43.26,78.56 42.13,78.56 v41.68,78.12 | v36.93,71.02 31.75,71.02 31.72,70.99
  GND 0.406: v35.64,76.23 v36.16,76.23 v36.17,76.22 v36.17,75.74 36.17,75.34 v36.14,75.31
  GND1 0.076: 34.98,75.01 34.98,75.16 v35.33,75.51
  GND1 0.102: U7.F4 36.55,75.11 | U7.N9 33.74,76.97 v33.45,76.68 | 33.55,74.6 33.35,74.4 v33.35,74.35 33.35,74.37 v33.55,74.57 | 34.52,73.94 34.98,74.4 34.98,74.95 34.98,75.01 | v35.33,75.51
  GND1 0.152: v36.96,74.6 36.96,74.75 37.01,74.8 37.01,74.91 | v32.23,72.41 32.23,72.35 32.74,71.84
  GND1 0.203: U7.F4 | v35.33,75.51 35.33,75.97 35.43,76.07
  GND1 0.254: v39.8,76.66 39.8,76.4 v39.88,76.33 | 33.07,77.93 32.94,78.05 | 32.94,78.05 32.03,78.97 | 32.94,78.05 32.94,78 | 33,77.95 32.94,78 | 32.94,78 34.06,78 U7.M11 | v42.24,72.29 42.01,72.29 v41.81,72.49 41.5,72.8 v41.48,72.8 | v44.04,74.35 44.17,74.35 X3.4 44.7,74.88 v44.81,74.88 | v33.58,73.05 34.06,73.05 34.98,73.96 34.98,74.95
  GND1 0.305: U7.M11 | U7.M11
  GND1 0.508: 37.77,74.02 36.37,75.41 36.37,76.02 v36.17,76.22
  Bottom 0.076: U1.B3 55.01,80.29 55.01,79.9 54.74,79.63 | U1.J9 58.01,84.3 58.5,84.3 58.55,84.35 58.55,84.4 58.6,84.45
